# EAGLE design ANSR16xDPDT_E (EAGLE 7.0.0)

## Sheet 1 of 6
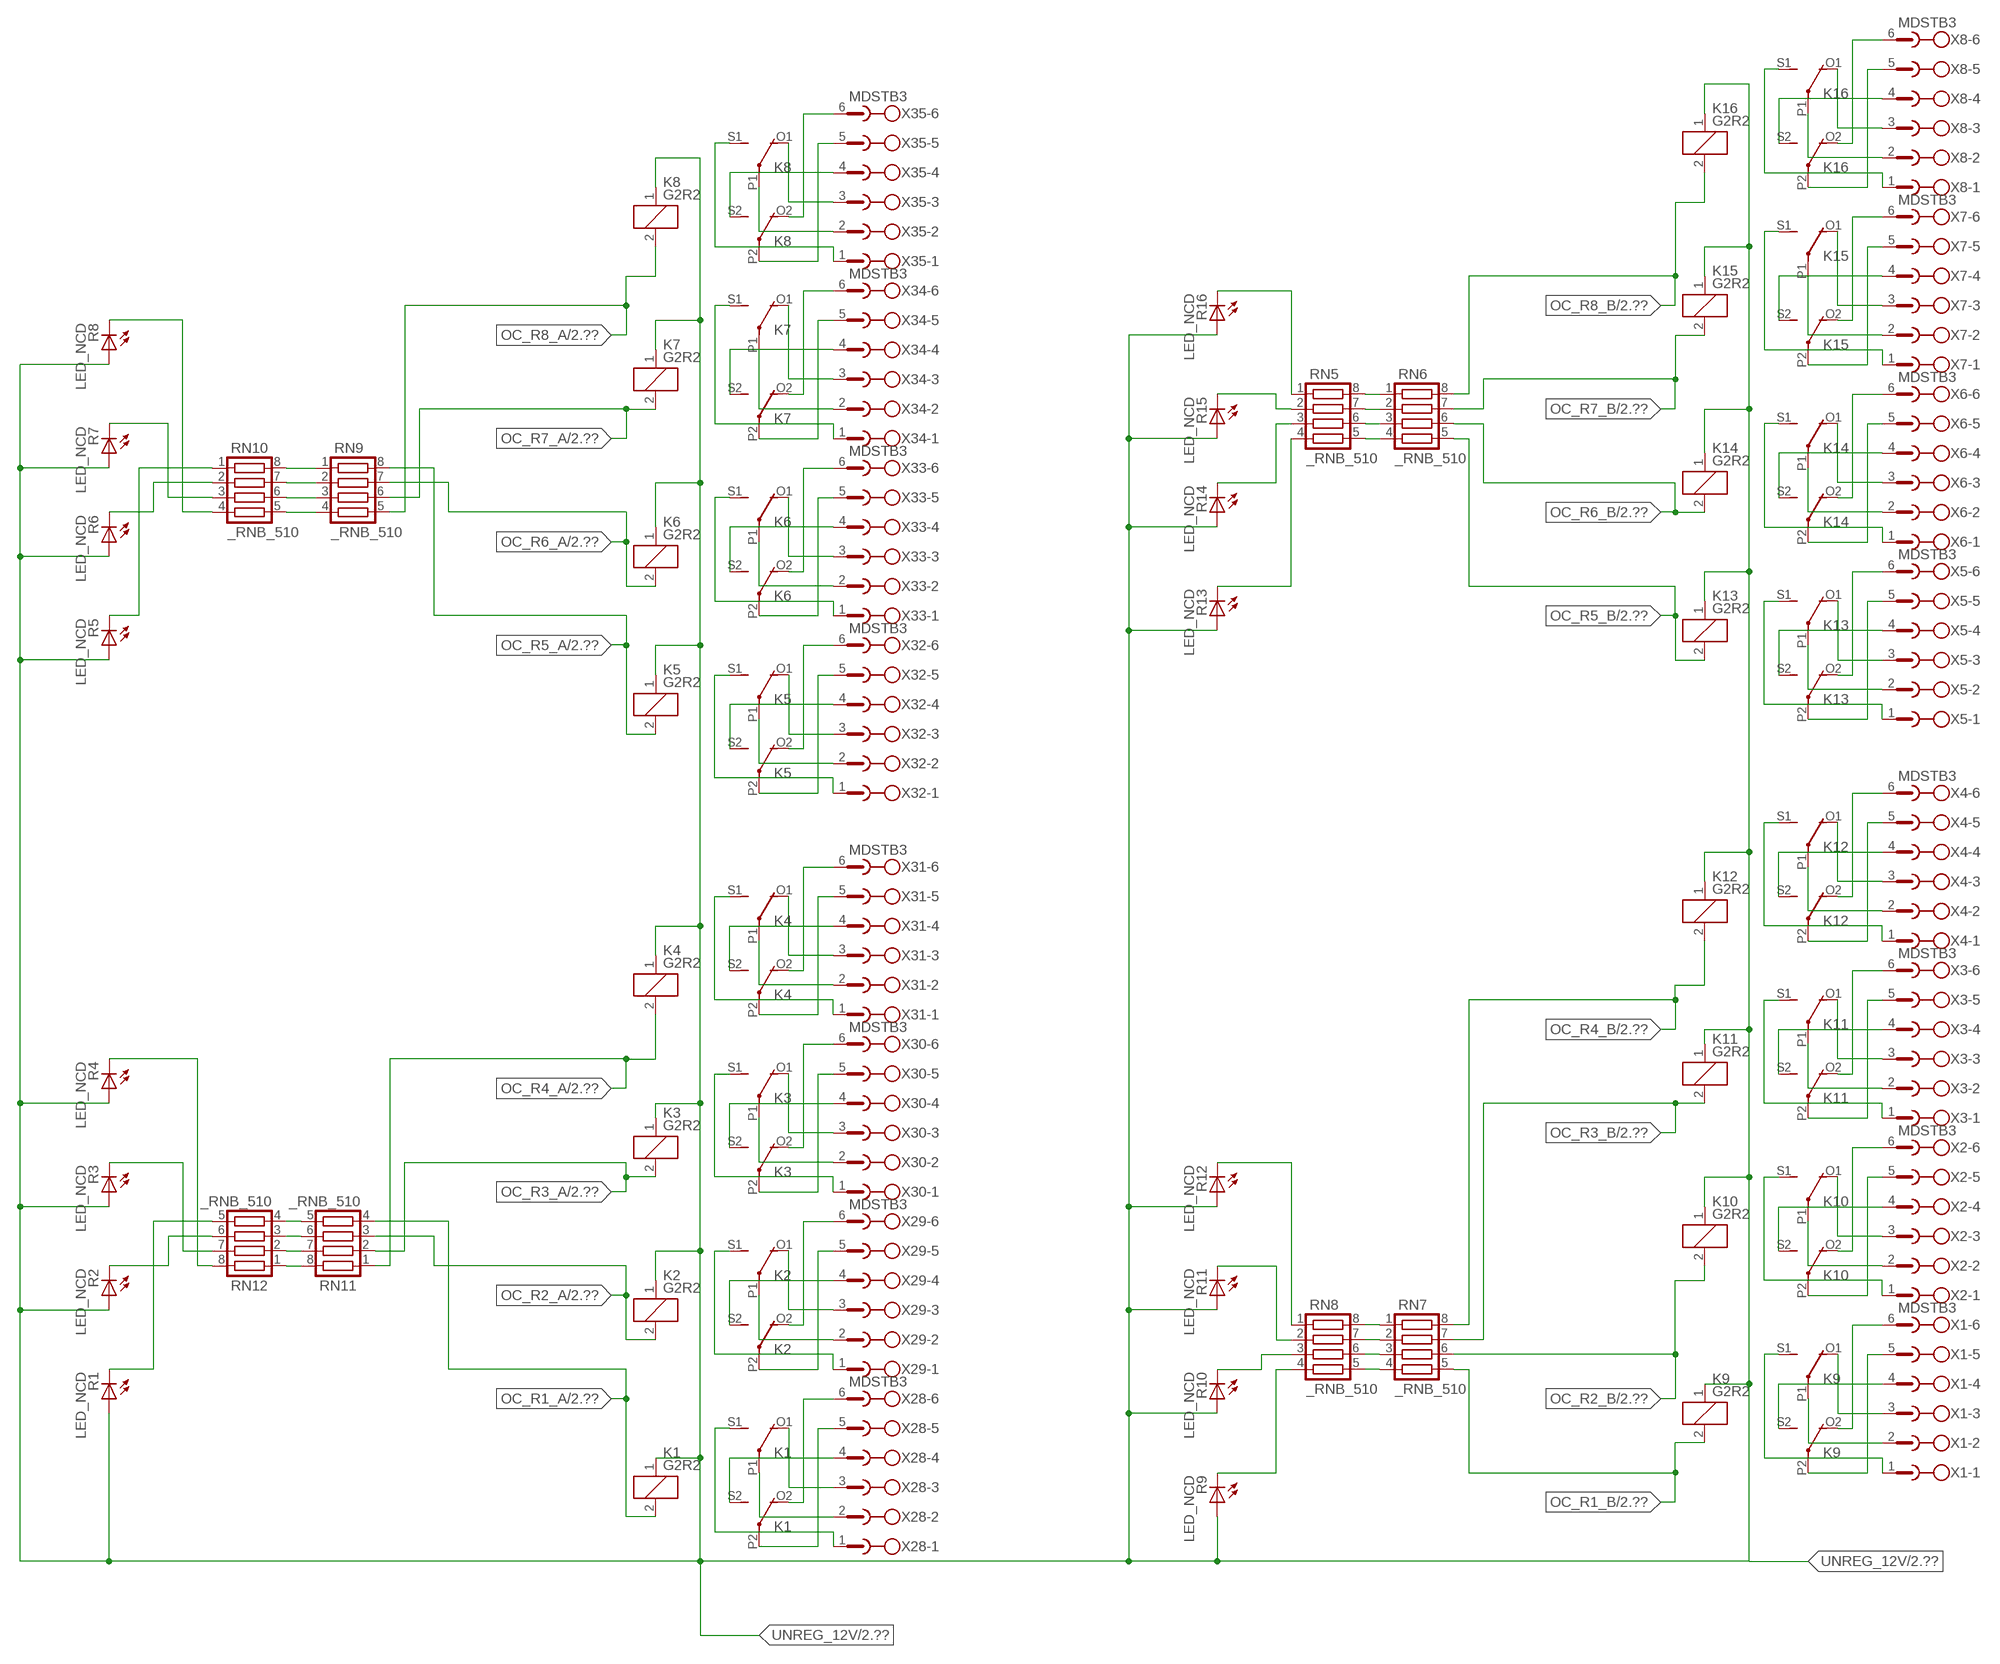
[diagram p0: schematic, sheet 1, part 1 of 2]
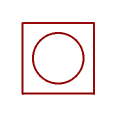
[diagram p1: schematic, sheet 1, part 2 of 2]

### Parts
K1  G2R2  [G2R2]
K2  G2R2  [G2R2]
K3  G2R2  [G2R2]
K4  G2R2  [G2R2]
K5  G2R2  [G2R2]
K6  G2R2  [G2R2]
K7  G2R2  [G2R2]
K8  G2R2  [G2R2]
K9  G2R2  [G2R2]
K10  G2R2  [G2R2]
K11  G2R2  [G2R2]
K12  G2R2  [G2R2]
K13  G2R2  [G2R2]
K14  G2R2  [G2R2]
K15  G2R2  [G2R2]
K16  G2R2  [G2R2]
R1  LED_NCD  [CHIPLED_0603]
R2  LED_NCD  [CHIPLED_0603]
R3  LED_NCD  [CHIPLED_0603]
R4  LED_NCD  [CHIPLED_0603]
R5  LED_NCD  [CHIPLED_0603]
R6  LED_NCD  [CHIPLED_0603]
R7  LED_NCD  [CHIPLED_0603]
R8  LED_NCD  [CHIPLED_0603]
R9  LED_NCD  [CHIPLED_0603]
R10  LED_NCD  [CHIPLED_0603]
R11  LED_NCD  [CHIPLED_0603]
R12  LED_NCD  [CHIPLED_0603]
R13  LED_NCD  [CHIPLED_0603]
R14  LED_NCD  [CHIPLED_0603]
R15  LED_NCD  [CHIPLED_0603]
R16  LED_NCD  [CHIPLED_0603]
RN5  _RNB_510  [RNB]
RN6  _RNB_510  [RNB]
RN7  _RNB_510  [RNB]
RN8  _RNB_510  [RNB]
RN9  _RNB_510  [RNB]
RN10  _RNB_510  [RNB]
RN11  _RNB_510  [RNB]
RN12  _RNB_510  [RNB]
U$1  PCB_MOUNTING_HOLE  [PCB_MOUNTING_HOLE]
X1  MDSTB3  [MDSTB3]
X2  MDSTB3  [MDSTB3]
X3  MDSTB3  [MDSTB3]
X4  MDSTB3  [MDSTB3]
X5  MDSTB3  [MDSTB3]
X6  MDSTB3  [MDSTB3]
X7  MDSTB3  [MDSTB3]
X8  MDSTB3  [MDSTB3]
X28  MDSTB3  [MDSTB3]
X29  MDSTB3  [MDSTB3]
X30  MDSTB3  [MDSTB3]
X31  MDSTB3  [MDSTB3]
X32  MDSTB3  [MDSTB3]
X33  MDSTB3  [MDSTB3]
X34  MDSTB3  [MDSTB3]
X35  MDSTB3  [MDSTB3]

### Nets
N$1: K9.P2(3:COM) X1.5
N$2: K9.O2(3:NC) X1.6
N$3: K9.S2(3:NO) X1.4
N$4: K9.P1(2:COM) X1.2
N$5: K9.O1(2:NC) X1.3
N$6: K9.S1(2:NO) X1.1
N$7: K10.P2(3:COM) X2.5
N$8: K10.O2(3:NC) X2.6
N$9: K10.S2(3:NO) X2.4
N$10: K10.S1(2:NO) X2.1
N$11: K10.P1(2:COM) X2.2
N$12: K10.O1(2:NC) X2.3
N$13: K11.P2(3:COM) X3.5
N$14: K11.O2(3:NC) X3.6
N$15: K12.P2(3:COM) X4.5
N$16: K12.O2(3:NC) X4.6
N$17: K11.S2(3:NO) X3.4
N$18: K12.S2(3:NO) X4.4
N$19: K11.O1(2:NC) X3.3
N$20: K12.O1(2:NC) X4.3
N$21: K12.P1(2:COM) X4.2
N$22: K11.P1(2:COM) X3.2
N$23: K11.S1(2:NO) X3.1
N$24: K12.S1(2:NO) X4.1
N$25: K13.O2(3:NC) X5.6
N$26: K13.P2(3:COM) X5.5
N$27: K13.S2(3:NO) X5.4
N$28: K13.P1(2:COM) X5.2
N$29: K13.S1(2:NO) X5.1
N$30: K13.O1(2:NC) X5.3
N$31: K14.P2(3:COM) X6.5
N$32: K14.O2(3:NC) X6.6
N$33: K14.P1(2:COM) X6.2
N$34: K14.S1(2:NO) X6.1
N$35: K15.P1(2:COM) X7.2
N$36: K16.P1(2:COM) X8.2
N$37: K16.P2(3:COM) X8.5
N$38: K16.O2(3:NC) X8.6
N$39: K14.O1(2:NC) X6.3
N$40: K16.O1(2:NC) X8.3
N$41: K15.O1(2:NC) X7.3
N$42: K15.O2(3:NC) X7.6
N$43: K15.P2(3:COM) X7.5
N$44: K14.S2(3:NO) X6.4
N$45: K15.S2(3:NO) X7.4
N$46: K15.S1(2:NO) X7.1
N$47: K16.S1(2:NO) X8.1
N$48: K16.S2(3:NO) X8.4
N$203: K1.P2(3:COM) X28.5
N$204: K1.O2(3:NC) X28.6
N$205: K1.S2(3:NO) X28.4
N$206: K1.P1(2:COM) X28.2
N$207: K1.O1(2:NC) X28.3
N$208: K1.S1(2:NO) X28.1
N$209: K2.P2(3:COM) X29.5
N$210: K2.O2(3:NC) X29.6
N$211: K2.S2(3:NO) X29.4
N$212: K2.S1(2:NO) X29.1
N$213: K2.P1(2:COM) X29.2
N$214: K2.O1(2:NC) X29.3
N$215: K3.P2(3:COM) X30.5
N$216: K3.O2(3:NC) X30.6
N$217: K4.P2(3:COM) X31.5
N$218: K4.O2(3:NC) X31.6
N$219: K3.S2(3:NO) X30.4
N$220: K4.S2(3:NO) X31.4
N$221: K3.O1(2:NC) X30.3
N$222: K4.O1(2:NC) X31.3
N$223: K4.P1(2:COM) X31.2
N$224: K3.P1(2:COM) X30.2
N$225: K3.S1(2:NO) X30.1
N$226: K4.S1(2:NO) X31.1
N$304: K5.O2(3:NC) X32.6
N$305: K5.P2(3:COM) X32.5
N$306: K5.S2(3:NO) X32.4
N$307: K5.P1(2:COM) X32.2
N$308: K5.S1(2:NO) X32.1
N$309: K5.O1(2:NC) X32.3
N$310: K6.P2(3:COM) X33.5
N$311: K6.O2(3:NC) X33.6
N$312: K6.P1(2:COM) X33.2
N$313: K6.S1(2:NO) X33.1
N$314: K7.P1(2:COM) X34.2
N$315: K8.P1(2:COM) X35.2
N$316: K8.P2(3:COM) X35.5
N$317: K8.O2(3:NC) X35.6
N$318: K6.O1(2:NC) X33.3
N$319: K8.O1(2:NC) X35.3
N$320: K7.O1(2:NC) X34.3
N$321: K7.O2(3:NC) X34.6
N$322: K7.P2(3:COM) X34.5
N$323: K6.S2(3:NO) X33.4
N$324: K7.S2(3:NO) X34.4
N$325: K7.S1(2:NO) X34.1
N$326: K8.S1(2:NO) X35.1
N$327: K8.S2(3:NO) X35.4
N$441: R16.C RN5.1
N$442: RN7.2 RN8.7
N$443: RN7.3 RN8.6
N$444: RN7.4 RN8.5
N$445: R15.C RN5.2
N$447: R13.C RN5.4
N$448: RN5.5 RN6.4
N$449: RN7.1 RN8.8
N$450: R12.C RN8.1
N$451: RN5.6 RN6.3
N$452: R11.C RN8.2
N$453: RN5.7 RN6.2
N$454: RN5.8 RN6.1
N$458: R14.C RN5.3
N$459: R10.C RN8.3
N$463: RN11.5 RN12.4
N$470: R9.C RN8.4
N$473: R1.C RN12.5
N$474: RN11.6 RN12.3
N$475: R2.C RN12.6
N$476: R3.C RN12.7
N$477: RN9.4 RN10.5
N$478: RN9.3 RN10.6
N$479: RN9.2 RN10.7
N$480: RN9.1 RN10.8
N$481: RN11.7 RN12.2
N$482: R5.C RN10.1
N$483: R4.C RN12.8
N$484: R7.C RN10.3
N$485: R8.C RN10.4
N$486: R6.C RN10.2
N$500: RN11.8 RN12.1
OC_R1_A: K1.2(1:C2) RN11.4 ; also sheet 2
OC_R1_B: K9.2(1:C2) RN7.5 ; also sheet 2
OC_R2_A: K2.2(1:C2) RN11.3 ; also sheet 2
OC_R2_B: K10.2(1:C2) RN7.6 ; also sheet 2
OC_R3_A: K3.2(1:C2) RN11.2 ; also sheet 2
OC_R3_B: K11.2(1:C2) RN7.7 ; also sheet 2
OC_R4_A: K4.2(1:C2) RN11.1 ; also sheet 2
OC_R4_B: K12.2(1:C2) RN7.8 ; also sheet 2
OC_R5_A: K5.2(1:C2) RN9.8 ; also sheet 2
OC_R5_B: K13.2(1:C2) RN6.5 ; also sheet 2
OC_R6_A: K6.2(1:C2) RN9.7 ; also sheet 2
OC_R6_B: K14.2(1:C2) RN6.6 ; also sheet 2
OC_R7_A: K7.2(1:C2) RN9.6 ; also sheet 2
OC_R7_B: K15.2(1:C2) RN6.7 ; also sheet 2
OC_R8_A: K8.2(1:C2) RN9.5 ; also sheet 2
OC_R8_B: K16.2(1:C2) RN6.8 ; also sheet 2
UNREG_12V: K1.1(1:C1) K2.1(1:C1) K3.1(1:C1) K4.1(1:C1) K5.1(1:C1) K6.1(1:C1) K7.1(1:C1) K8.1(1:C1) K9.1(1:C1) K10.1(1:C1) K11.1(1:C1) K12.1(1:C1) K13.1(1:C1) K14.1(1:C1) K15.1(1:C1) K16.1(1:C1) R1.A R2.A R3.A R4.A R5.A R6.A R7.A R8.A R9.A R10.A R11.A R12.A R13.A R14.A R15.A R16.A ; also sheet 2,3

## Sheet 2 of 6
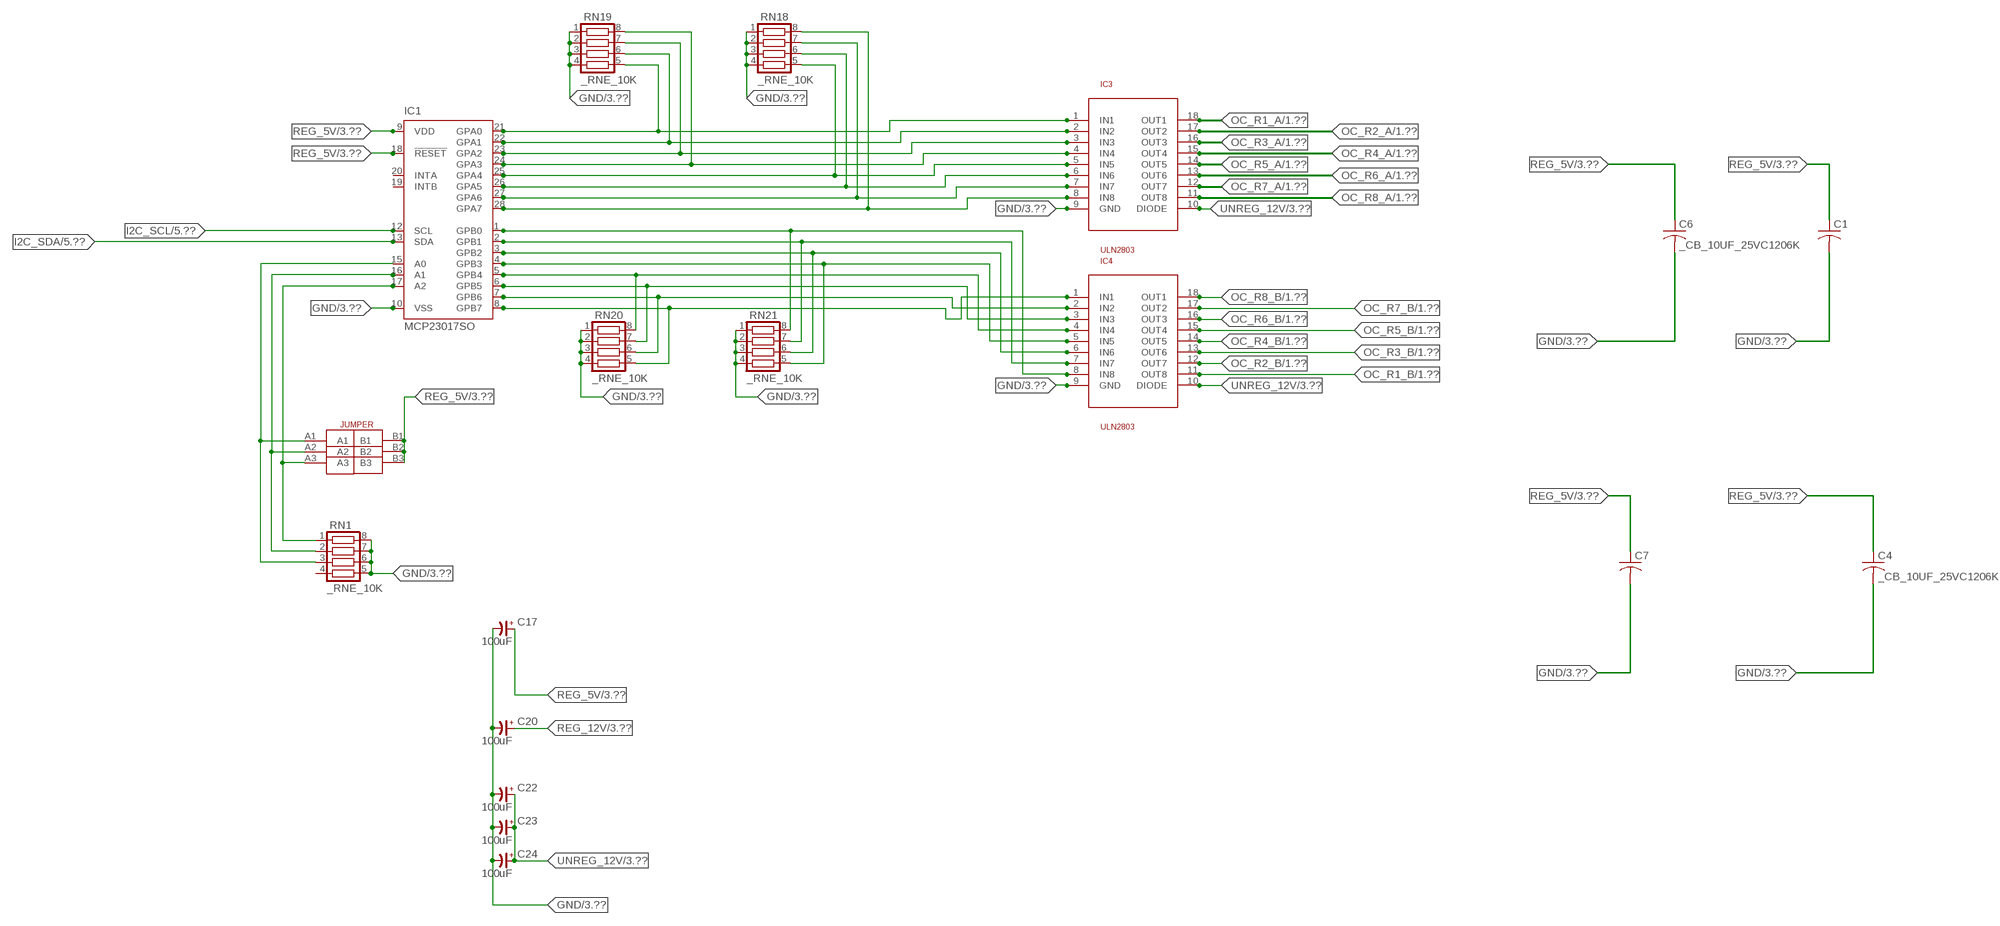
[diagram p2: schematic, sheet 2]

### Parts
C1  _CA_.10UF_50VC1206K  [_CA_.1UF_50V]
C4  _CB_10UF_25VC1206K  [_CB_10UF_25V]
C6  _CB_10UF_25VC1206K  [_CB_10UF_25V]
C7  _CA_.10UF_50VC1206K  [_CA_.1UF_50V]
C17  100uF  CP-E-025X060  [E-025X060]
C20  100uF  CP-E-025X060  [E-025X060]
C22  100uF  CP-E-025X060  [E-025X060]
C23  100uF  CP-E-025X060  [E-025X060]
C24  100uF  CP-E-025X060  [E-025X060]
IC1  MCP23017SO  [SO28W]
IC3  ULN2803  [SO18L]
IC4  ULN2803  [SO18L]
JP1  JUMPER_3X2  [JUMPER_3X2]
RN1  _RNE_10K  [RNE]
RN18  _RNE_10K  [RNE]
RN19  _RNE_10K  [RNE]
RN20  _RNE_10K  [RNE]
RN21  _RNE_10K  [RNE]

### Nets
GND: C1.2 C4.2 C6.2 C7.2 C17.- C20.- C22.- C23.- C24.- IC1.10(VSS) IC3.9(GND) IC4.9(GND) RN1.5 RN1.6 RN1.7 RN1.8 RN18.1 RN18.2 RN18.3 RN18.4 RN19.1 RN19.2 RN19.3 RN19.4 RN20.1 RN20.2 RN20.3 RN20.4 RN21.1 RN21.2 RN21.3 RN21.4 ; also sheet 3,4,5,6
I2C_SCL: IC1.12(SCL) ; also sheet 5,6
I2C_SDA: IC1.13(SDA) ; also sheet 5,6
N$49: IC1.15(A0) JP1.A1 RN1.3
N$405: IC1.21(GPA0) IC3.1(IN1) RN19.5
N$406: IC1.25(GPA4) IC3.5(IN5) RN18.5
N$407: IC1.26(GPA5) IC3.6(IN6) RN18.6
N$408: IC1.16(A1) JP1.A2 RN1.2
N$409: IC1.22(GPA1) IC3.2(IN2) RN19.6
N$410: IC1.23(GPA2) IC3.3(IN3) RN19.7
N$411: IC1.24(GPA3) IC3.4(IN4) RN19.8
N$416: IC1.1(GPB0) IC4.8(IN8) RN21.8
N$417: IC1.2(GPB1) IC4.7(IN7) RN21.7
N$418: IC1.3(GPB2) IC4.6(IN6) RN21.6
N$419: IC1.4(GPB3) IC4.5(IN5) RN21.5
N$420: IC1.5(GPB4) IC4.4(IN4) RN20.8
N$421: IC1.6(GPB5) IC4.3(IN3) RN20.7
N$422: IC1.7(GPB6) IC4.2(IN2) RN20.6
N$423: IC1.8(GPB7) IC4.1(IN1) RN20.5
N$498: IC1.17(A2) JP1.A3 RN1.1
N$525: IC1.27(GPA6) IC3.7(IN7) RN18.7
N$526: IC1.28(GPA7) IC3.8(IN8) RN18.8
OC_R1_A: IC3.18(OUT1) ; also sheet 1
OC_R1_B: IC4.11(OUT8) ; also sheet 1
OC_R2_A: IC3.17(OUT2) ; also sheet 1
OC_R2_B: IC4.12(OUT7) ; also sheet 1
OC_R3_A: IC3.16(OUT3) ; also sheet 1
OC_R3_B: IC4.13(OUT6) ; also sheet 1
OC_R4_A: IC3.15(OUT4) ; also sheet 1
OC_R4_B: IC4.14(OUT5) ; also sheet 1
OC_R5_A: IC3.14(OUT5) ; also sheet 1
OC_R5_B: IC4.15(OUT4) ; also sheet 1
OC_R6_A: IC3.13(OUT6) ; also sheet 1
OC_R6_B: IC4.16(OUT3) ; also sheet 1
OC_R7_A: IC3.12(OUT7) ; also sheet 1
OC_R7_B: IC4.17(OUT2) ; also sheet 1
OC_R8_A: IC3.11(OUT8) ; also sheet 1
OC_R8_B: IC4.18(OUT1) ; also sheet 1
REG_5V: C1.1 C4.1 C6.1 C7.1 C17.+ IC1.9(VDD) IC1.18(!RESET) JP1.B1 JP1.B2 JP1.B3 ; also sheet 3,4,5,6
REG_12V: C20.+ ; also sheet 3,4
UNREG_12V: C22.+ C23.+ C24.+ IC3.10(DIODE) IC4.10(DIODE) ; also sheet 1,3
Unconnected: IC1.19(INTB) IC1.20(INTA) RN1.4

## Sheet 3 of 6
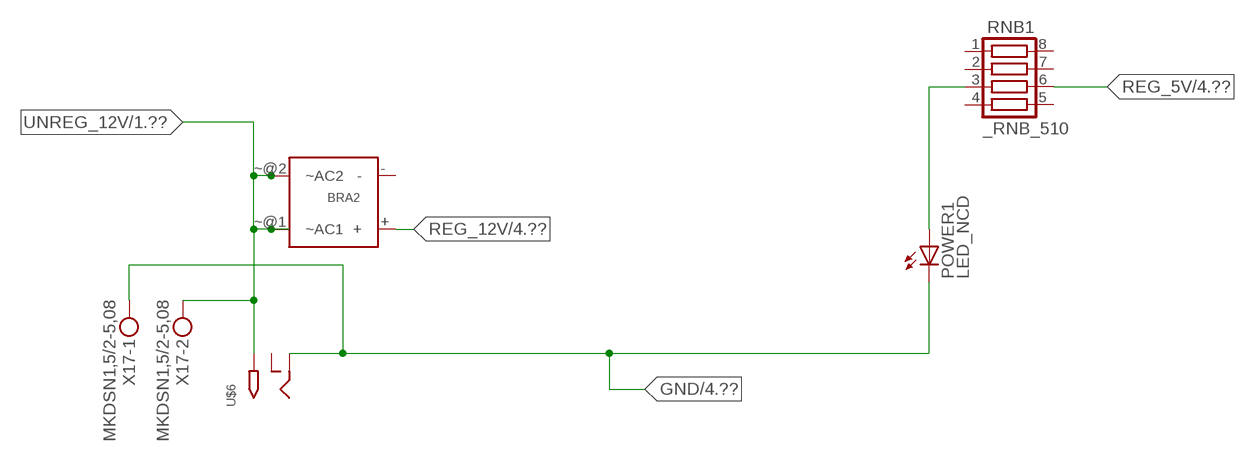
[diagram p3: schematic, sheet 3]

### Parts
BRA2  MB2S_  [MB2S]
POWER1  LED_NCD  [CHIPLED_0603]
RNB1  _RNB_510  [RNB]
U$6  2.1MMJACK  [PJ-102A]
X17  MKDSN1,5/2-5,08  [MKDSN1,5/2-5,08]

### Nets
GND: POWER1.C U$6.RING X17.1 ; also sheet 2,4,5,6
N$99: POWER1.A RNB1.3
REG_5V: RNB1.6 ; also sheet 2,4,5,6
REG_12V: BRA2.+ ; also sheet 2,4
UNREG_12V: BRA2.~@1(~AC1) BRA2.~@2(~AC2) U$6.TIP X17.2 ; also sheet 1,2
Unconnected: BRA2.- RNB1.1 RNB1.2 RNB1.4 RNB1.5 RNB1.7 RNB1.8 U$6.RING_SW

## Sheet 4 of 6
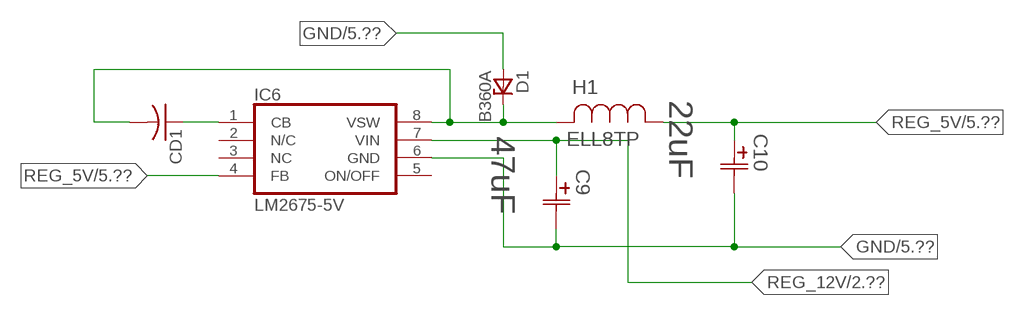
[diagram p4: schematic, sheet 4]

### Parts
C9  47uF  490-5463-6-NDCAP  [C2917(7343)-Y]
C10  22uF  490-5463-6-NDCAP  [C2917(7343)-Y]
CD1  _CD_10NF_50VC1206K  [_CD_10NF_50V]
D1  B360A  [DO214AC_ZENER]
H1  ELL8TP  [IND_ELL8TP]
IC6  LM2675-5V  LM2675  [SO-8]

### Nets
GND: C9.2(C2) C10.2(C2) D1.A IC6.6(GND) ; also sheet 2,3,5,6
N$100: CD1.2 D1.C H1.2 IC6.8(VSW)
N$101: CD1.1 IC6.1(CB)
REG_5V: C10.1(C1) H1.1 IC6.4(FB) ; also sheet 2,3,5,6
REG_12V: C9.1(C1) IC6.7(VIN) ; also sheet 2,3
Unconnected: IC6.2(N/C) IC6.5(ON/OFF)

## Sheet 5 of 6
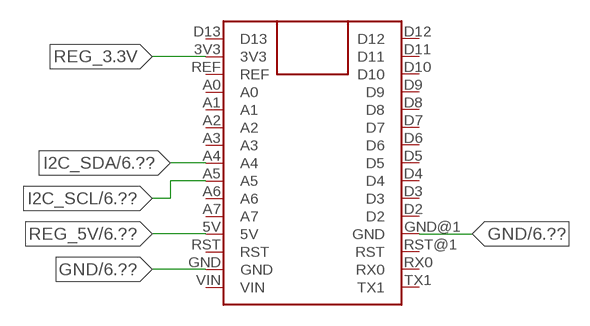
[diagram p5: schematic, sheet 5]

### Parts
FOR_NANO  ARDUINO_NANO  [ARDUINO_NANO]

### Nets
GND: FOR_NANO.GND FOR_NANO.GND@1(GND) ; also sheet 2,3,4,6
I2C_SCL: FOR_NANO.A5 ; also sheet 2,6
I2C_SDA: FOR_NANO.A4 ; also sheet 2,6
REG_3.3V: FOR_NANO.3V3
REG_5V: FOR_NANO.5V ; also sheet 2,3,4,6
Unconnected: FOR_NANO.A0 FOR_NANO.A1 FOR_NANO.A2 FOR_NANO.A3 FOR_NANO.A6 FOR_NANO.A7 FOR_NANO.D2 FOR_NANO.D3 FOR_NANO.D4 FOR_NANO.D5 FOR_NANO.D6 FOR_NANO.D7 FOR_NANO.D8 FOR_NANO.D9 FOR_NANO.D10 FOR_NANO.D11 FOR_NANO.D12 FOR_NANO.D13 FOR_NANO.REF FOR_NANO.RST FOR_NANO.RST@1(RST) FOR_NANO.RX0 FOR_NANO.TX1 FOR_NANO.VIN

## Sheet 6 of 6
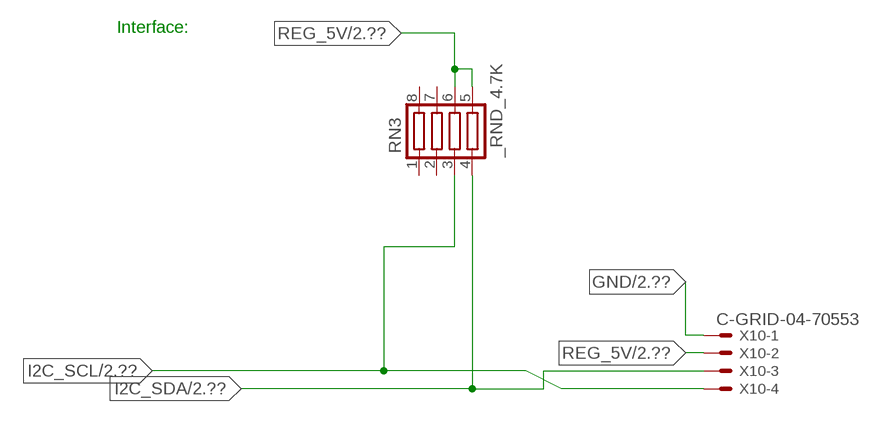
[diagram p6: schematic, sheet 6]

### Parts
RN3  _RND_4.7K  [RND]
X10  C-GRID-04-70553  [70553-04]

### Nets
GND: X10.1 ; also sheet 2,3,4,5
I2C_SCL: RN3.3 X10.4 ; also sheet 2,5
I2C_SDA: RN3.4 X10.3 ; also sheet 2,5
REG_5V: RN3.5 RN3.6 X10.2 ; also sheet 2,3,4,5
Unconnected: RN3.1 RN3.2 RN3.7 RN3.8

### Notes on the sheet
- Interface:

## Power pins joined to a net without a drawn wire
NC: IC6.3(NC)

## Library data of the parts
BRA2 = NCD_ULTIMATE_LIBRARY:MB2S: Bridge Rectifier BRA MB2S 200V 500ma Digikey MB2S-TPMSTR-ND/MB2S-TP
C1 C7 = NCD_ULTIMATE_LIBRARY:_CA_.10UF_50V: Capacitor .1uF SMT
C4 C6 = NCD_ULTIMATE_LIBRARY:_CB_10UF_25V: Capacitor 10uF SMT
C9 C10 = NCD_ULTIMATE_bhaskar:490-5463-6-ND: NCD CAP
C17 C20 C22-C24 = NCD_ULTIMATE_LIBRARY:CP-: Capacitors All Kinds POLARIZED CAP
CD1 = NCD_ULTIMATE_LIBRARY:_CD_10NF_50V: Capacitor 10nF SMT
D1 = NCD_ULTIMATE_bhaskar:B360A: NCD DIODE B350A/B360A
FOR_NANO = NCD_ULTIMATE_CONNECTORS:ARDUINO_NANO
H1 = NCD_ULTIMATE_bhaskar:ELL8TP: NCD coil
IC1 = NCD_ULTIMATE_LIBRARY:MCP23017: Semiconductor Port Expander I/O 16-Bit I2C http://ww1.microchip.com/downloads/en/DeviceDoc/21952a.pdf Source: http://ww1.microchip.com/downloads/en/DeviceDoc/21952a.pdf
IC3 IC4 = NCD_ULTIMATE_LIBRARY:ULN2803: Semiconductor 8 O.C. N-Channel Transistor Driver Digikey ULN2803AFWGCELTR-ND/ULN2803AFWG,C,EL
IC6 = NCD_ULTIMATE_bhaskar:LM2675: LM2675 NCD http://www.ti.com/lit/ds/symlink/lm2675.pdf
JP1 = NCD_ULTIMATE_CONNECTORS:JUMPER_3X2
K1-K16 = NCD_ULTIMATE_LIBRARY:G2R2: RELAY 2 x switch, Omron
POWER1 R1-R16 = NCD_ULTIMATE_bhaskar:LED_NCD
RN1 RN18-RN21 = NCD_ULTIMATE_LIBRARY:_RNE_10K: Resistor Array RNE SMT 10K x 4 Single Resistor Source: http://www.ctscorp.com/components/Datasheets/CTSChipArrayDs.pdf Digikey 742C083103JPTR-ND/742C083103JP; OC_FARNELL: unknown; OC_NEWARK: unknown
RN3 = NCD_ULTIMATE_LIBRARY:_RND_4.7K: Resistor Array RND SMT 4.7K x 4 Single Resistor Source: http://www.ctscorp.com/components/Datasheets/CTSChipArrayDs.pdf Digikey 742C083472JPTR-ND/742C083472JP; OC_FARNELL: unknown; OC_NEWARK: unknown
RN5-RN12 RNB1 = NCD_ULTIMATE_LIBRARY:_RNB_510: Resistor Array RNB SMT 510 x 4 Single Resistor Source: http://www.ctscorp.com/components/Datasheets/CTSChipArrayDs.pdf Digikey 742C083511JPTR-ND/ 742C083511JP; OC_FARNELL: unknown; OC_NEWARK: unknown
U$1 = NCD_ULTIMATE_CONNECTORS:PCB_MOUNTING_HOLE
U$6 = NCD_ULTIMATE_CONNECTORS:2.1MMJACK: 2.1mm x 5.5mm DC jack with internal switch. Digikey part #PJ-102A, 4UCON part #05537 By microbuilder.eu
X1-X8 X28-X35 = NCD_ULTIMATE_LIBRARY:MDSTB3: PHOENIX
X10 = NCD_ULTIMATE_CONNECTORS:C-GRID-04: CONNECTOR 4-Pos I2C wire to board 2.54 mm (0.100") pitch header Digikey WM1342-ND/0015912045; OC_FARNELL: unknown; OC_NEWARK: unknown
X17 = NCD_ULTIMATE_CONNECTORS:MKDSN1,5/2-5,08: MKDSN 1,5/ 2-5,08 Printklemme

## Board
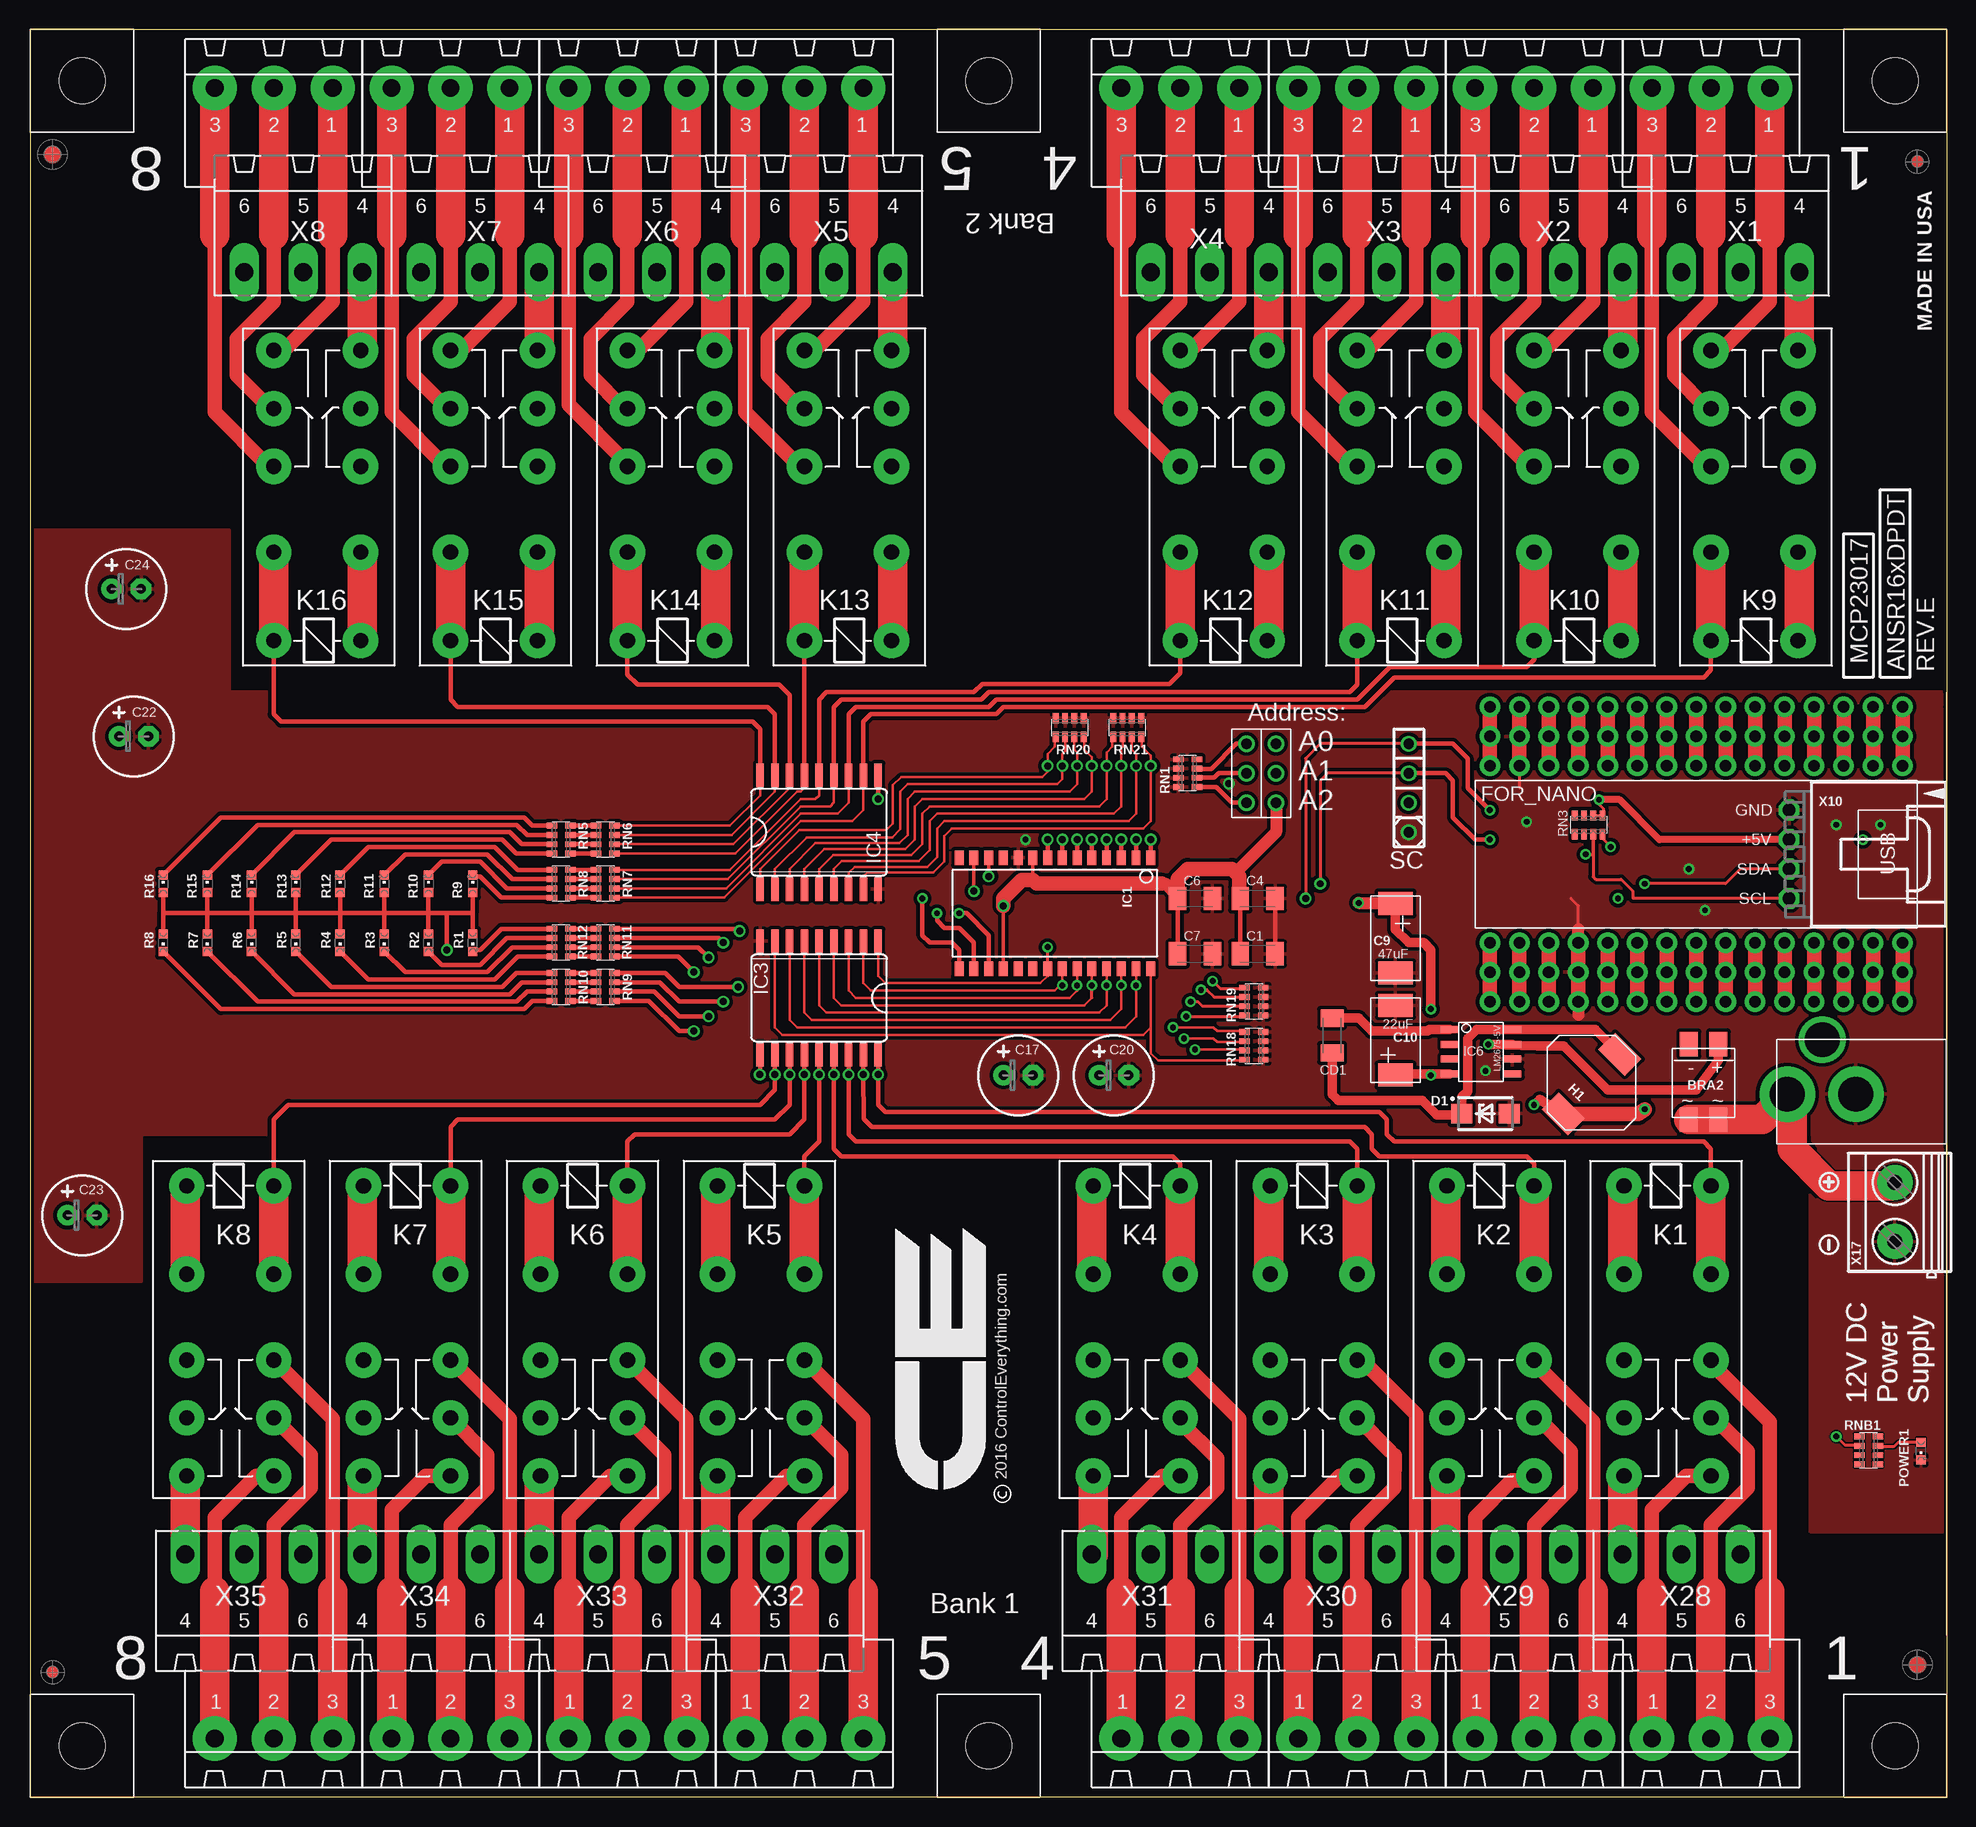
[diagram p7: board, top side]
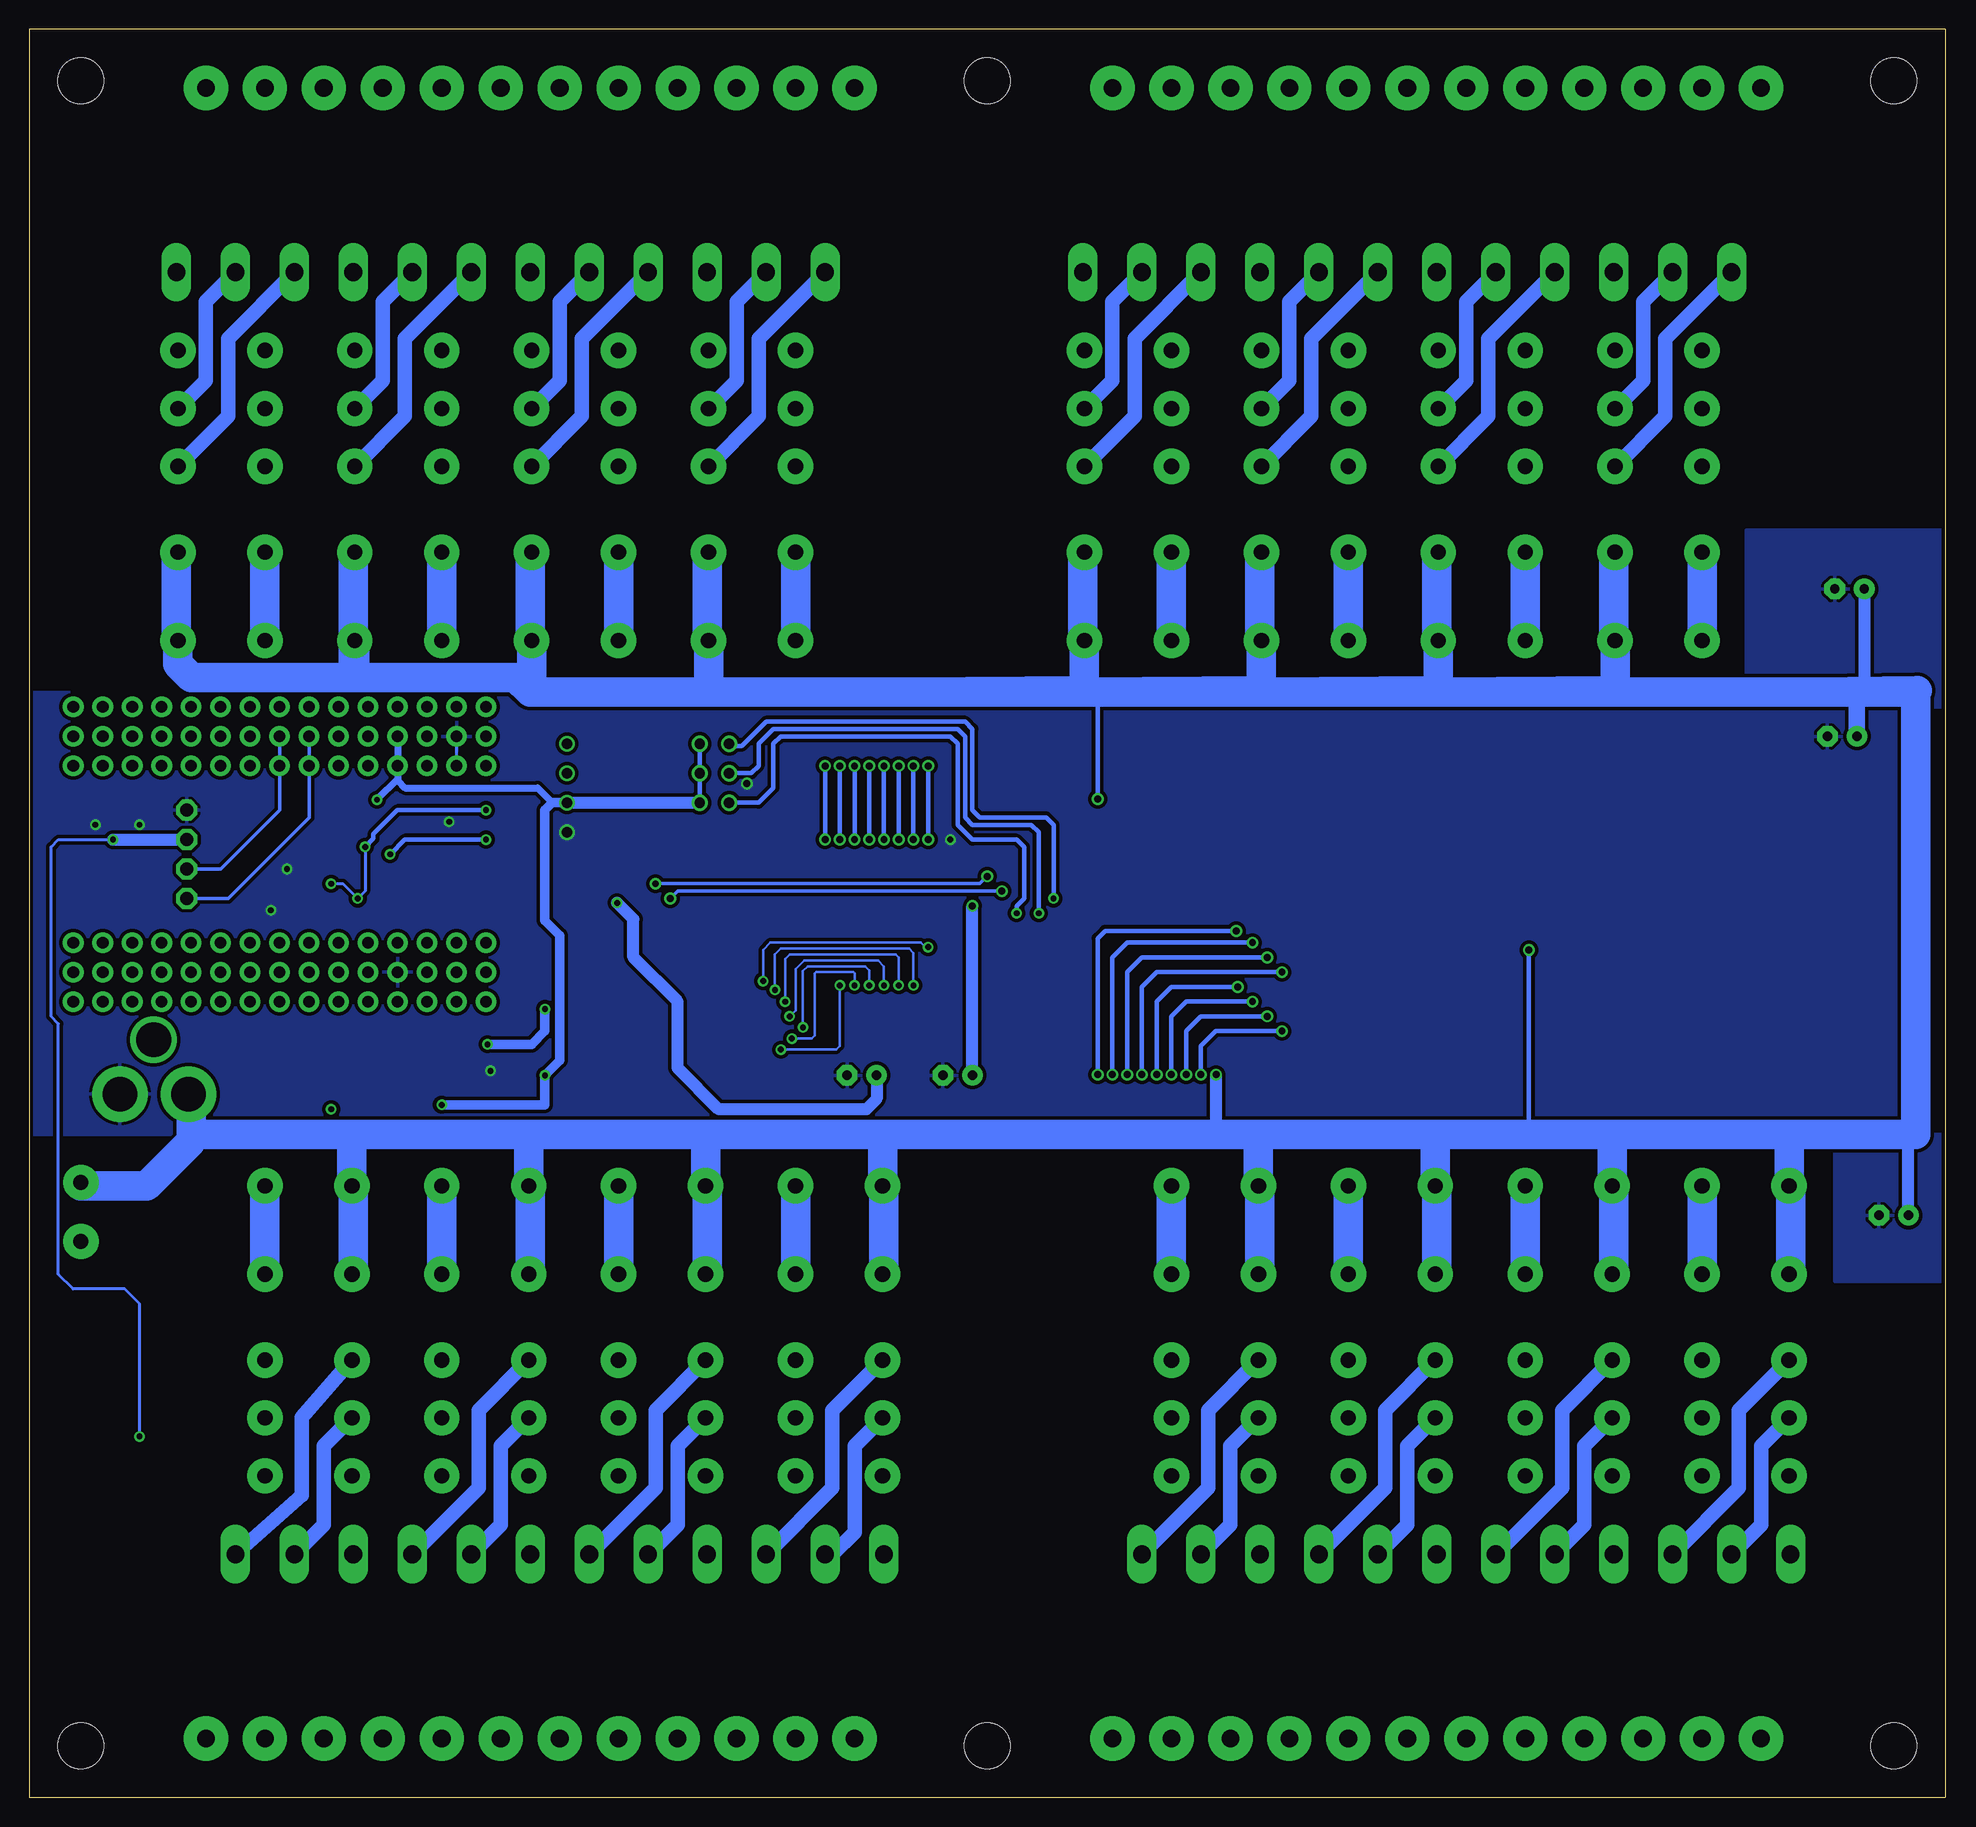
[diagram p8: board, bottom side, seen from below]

Size 165.1 x 152.41 mm. Coordinates in mm from the lower left corner, seen from the top.
Outline: 165.08,0 165.08,152.41 0,152.41 0,0.01 165.1,0.01
Outline: 165.08,93.99 165.08,13.97
Outline: 165.08,95.26 165.08,14.6
Outline: 165.1,95.26 165.1,37.48
Copper layers (1*16): Top 0.035mm / dielectric 1.5mm / Bottom 0.035mm
Design rules "default": minimum track width 5mil, minimum drill 24mil, track to track 5mil, track to pad 5mil, pad to pad 5mil, via to via 5mil, smd to smd 5mil, copper to edge 10mil, drill to drill 8mil, minimum pad ring 10mil, minimum via ring 8mil, stop-mask expansion 2mil, vias tented up to drill 0mil, thermal gap 10mil

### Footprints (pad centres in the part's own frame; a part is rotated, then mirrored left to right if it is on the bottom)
MB2S = smd 1.55 x 2.1: + 0,-6.5; - 2.54,-6.5; ~@1 0,0; ~@2 2.54,0
_CA_.1UF_50V = smd 1.5 x 2: 1 -1.5,0; 2 1.5,0
_CB_10UF_25V = smd 1.5 x 2: 1 -1.5,0; 2 1.5,0
C2917(7343)-Y = smd 2 x 3: 1 -3,0; 2 3,0
E-025X060 = drill 0.813 pad 1.778: + -1.27,0 | drill 0.813 pad 1.778 octagon: - 1.27,0
_CD_10NF_50V = smd 1.5 x 2: 1 -1.5,0; 2 1.5,0
DO214AC_ZENER = smd 1.8 x 1.7: A 2.05,0; C -2.05,0
ARDUINO_NANO = drill 1 pad 1.778: 3V1 -2.54,-2.54; 3V3 0,-2.54; 5V 0,-27.94; 5V1 -2.54,-27.94; A0 0,-7.62; A1 0,-10.16; A2 0,-12.7; A3 0,-15.24; A4 0,-17.78; A5 0,-20.32; A6 0,-22.86; A7 0,-25.4; A8 -2.54,-7.62; A9 -2.54,-10.16; A10 -2.54,-12.7; A11 -2.54,-15.24; A12 -2.54,-17.78; A13 -2.54,-20.32; A14 -2.54,-22.86; A15 -2.54,-25.4; D1 -2.54,0; D2 20.32,-25.4; D3 20.32,-22.86; D4 20.32,-20.32; D5 20.32,-17.78; D6 20.32,-15.24; D7 20.32,-12.7; D8 20.32,-10.16; D9 20.32,-7.62; D10 20.32,-5.08; D11 20.32,-2.54; D12 20.32,0; D13 0,0; D14 22.86,0; D15 22.86,-2.54; D16 22.86,-5.08; D17 22.86,-7.62; D18 22.86,-10.16; D19 22.86,-12.7; D20 22.86,-15.24; D21 22.86,-17.78; D22 22.86,-20.32; D23 22.86,-22.86; D24 22.86,-25.4; GND 0,-33.02; GND1 -2.54,-33.02; GND@1 20.32,-27.94; GND@2 22.86,-27.94; P$16 2.54,0; P$17 2.54,-2.54; P$18 2.54,-5.08; P$19 2.54,-7.62; P$20 2.54,-10.16; P$21 2.54,-12.7; P$22 2.54,-15.24; P$23 2.54,-17.78; P$24 2.54,-20.32; P$25 2.54,-22.86; P$26 2.54,-25.4; P$27 2.54,-27.94; P$28 2.54,-30.48; P$29 2.54,-33.02; P$30 2.54,-35.56; P$31 17.78,0; P$32 17.78,-2.54; P$33 17.78,-5.08; P$34 17.78,-7.62; P$35 17.78,-10.16; P$36 17.78,-12.7; P$37 17.78,-15.24; P$38 17.78,-17.78; P$39 17.78,-20.32; P$40 17.78,-22.86; P$41 17.78,-25.4; P$42 17.78,-27.94; P$43 17.78,-30.48; P$44 17.78,-33.02; P$45 17.78,-35.56; REF 0,-5.08; REF1 -2.54,-5.08; RST 0,-30.48; RST1 -2.54,-30.48; RST@1 20.32,-30.48; RST@2 22.86,-30.48; RX0 20.32,-33.02; RX1 22.86,-33.02; TX1 20.32,-35.56; TX2 22.86,-35.56; VIN 0,-35.56; VIN1 -2.54,-35.56
IND_ELL8TP = smd 2.054 x 3.2 rotated 45: 1 -2.442,-2.696; 2 2.442,2.442
SO28W = smd 0.762 x 1.27: 1 -7.62,-4.78; 2 -6.35,-4.78; 3 -5.08,-4.78; 4 -3.81,-4.78; 5 -2.54,-4.78; 6 -1.27,-4.78; 7 0,-4.78; 8 1.27,-4.78; 9 2.54,-4.78; 10 3.81,-4.78; 11 5.08,-4.78; 12 6.35,-4.78; 13 7.62,-4.78; 14 8.89,-4.78; 15 8.89,4.78; 16 7.62,4.78; 17 6.35,4.78; 18 5.08,4.78; 19 3.81,4.78; 20 2.54,4.78; 21 1.27,4.78; 22 0,4.78; 23 -1.27,4.78; 24 -2.54,4.78; 25 -3.81,4.78; 26 -5.08,4.78; 27 -6.35,4.78; 28 -7.62,4.78
SO18L = smd 0.66 x 2.032: 1 -5.08,-4.902; 2 -3.81,-4.902; 3 -2.54,-4.902; 4 -1.27,-4.902; 5 0,-4.902; 6 1.27,-4.902; 7 2.54,-4.902; 8 3.81,-4.902; 9 5.08,-4.902; 10 5.08,4.902; 11 3.81,4.902; 12 2.54,4.902; 13 1.27,4.902; 14 0,4.902; 15 -1.27,4.902; 16 -2.54,4.902; 17 -3.81,4.902; 18 -5.08,4.902
SO-8 = smd 0.6 x 1.55: 1 -1.905,-2.69; 2 -0.635,-2.69; 3 0.635,-2.69; 4 1.905,-2.69; 5 1.905,2.71; 6 0.635,2.71; 7 -0.635,2.71; 8 -1.905,2.71
JUMPER_3X2 = drill 0.9: A1 0,5.08; A2 0,2.54; A3 0,0; B1 2.54,5.08; B2 2.54,2.54; B3 2.54,0
G2R2 = drill 1.321 pad 3.048: 1 -2.54,-3.683; 2 -2.54,3.81; 3 5.08,-3.683; 4 5.08,3.81; O1 12.471,3.81; O2 12.471,-3.683; P1 17.45,3.81; P2 17.45,-3.683; S1 22.454,3.81; S2 22.454,-3.683
CHIPLED_0603 = smd 0.8 x 0.8: A 0,-0.75; C 0,0.75
RNE = smd 0.5 x 0.9: 1 -1.2,-0.8; 2 -0.4,-0.8; 3 0.4,-0.8; 4 1.2,-0.8; 5 1.2,0.8; 6 0.4,0.8; 7 -0.4,0.8; 8 -1.2,0.8
RND = smd 0.5 x 0.9: 1 -1.2,-0.8; 2 -0.4,-0.8; 3 0.4,-0.8; 4 1.2,-0.8; 5 1.2,0.8; 6 0.4,0.8; 7 -0.4,0.8; 8 -1.2,0.8
RNB = smd 0.5 x 0.9: 1 -1.2,-0.8; 2 -0.4,-0.8; 3 0.4,-0.8; 4 1.2,-0.8; 5 1.2,0.8; 6 0.4,0.8; 7 -0.4,0.8; 8 -1.2,0.8
PCB_MOUNTING_HOLE = hole 3.962: 4.445,4.445
PJ-102A = drill 3 pad 4.8: RING 0.1,-3.39; TIP 0.1,-9.29 | drill 3 pad 3.251: RING_SW -4.6,-6.29
MDSTB3 = drill 1.524 pad 3.81: 1 -3.81,-10.795; 2 1.27,-10.795; 3 6.35,-10.795 | drill 1.524 pad 2.54 long: 4 -6.35,5.08; 5 -1.27,5.08; 6 3.81,5.08
70553-04 = drill 1.1 pad 1.778 octagon: 1 -3.81,-7.62; 2 -1.27,-7.62; 3 1.27,-7.62; 4 3.81,-7.62
MKDSN1,5/2-5,08 = drill 1.3 pad 3.048: 1 -2.561,0.025; 2 2.519,0.025

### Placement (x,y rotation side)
BRA2  145.41,58.43 180 top
C1  105.73,72.72 0 top
C4  105.73,77.48 0 top
C6  100.33,77.48 0 top
C7  100.33,72.72 0 top
C9  117.6,74.05 270 top
C10  117.6,65.27 90 top
C17  85.09,62.24 0 top
C20  93.34,62.24 0 top
C22  8.89,91.45 0 top
C23  4.44,50.18 0 top
C24  8.25,104.15 0 top
CD1  112.14,65.67 270 top
D1  125.35,58.94 0 top
FOR_NANO  161.29,91.45 270 top
H1  134.49,61.61 0 top
IC1  88.9,76.21 180 top
IC3  67.94,68.91 180 top
IC4  67.94,83.2 0 top
IC6  124.97,64.27 270 top
JP1  104.78,85.74 0 top
K1  140.97,50.18 270 top
K2  125.73,50.18 270 top
K3  110.49,50.18 270 top
K4  95.25,50.18 270 top
K5  62.86,50.18 270 top
K6  47.62,50.18 270 top
K7  32.38,50.18 270 top
K8  17.14,50.18 270 top
K9  148.59,102.25 90 top
K10  133.35,102.25 90 top
K11  118.11,102.25 90 top
K12  102.87,102.25 90 top
K13  70.48,102.25 90 top
K14  55.25,102.25 90 top
K15  40,102.25 90 top
K16  24.76,102.25 90 top
POWER1  162.88,29.86 180 top
R1  38.1,73.67 180 top
R2  34.29,73.67 180 top
R3  30.48,73.67 180 top
R4  26.67,73.67 180 top
R5  22.86,73.67 180 top
R6  19.05,73.67 180 top
R7  15.24,73.67 180 top
R8  11.43,73.67 180 top
R9  38.1,78.75 0 top
R10  34.29,78.75 0 top
R11  30.48,78.75 0 top
R12  26.67,78.75 0 top
R13  22.86,78.75 0 top
R14  19.05,78.75 0 top
R15  15.24,78.75 0 top
R16  11.43,78.75 0 top
RN1  99.69,88.28 90 top
RN3  134.24,83.83 0 top
RN5  45.72,82.56 270 top
RN6  49.53,82.56 270 top
RN7  49.53,78.75 270 top
RN8  45.72,78.75 270 top
RN9  49.53,69.86 270 top
RN10  45.72,69.86 270 top
RN11  49.53,73.67 90 top
RN12  45.72,73.67 90 top
RN18  105.41,64.78 90 top
RN19  105.41,68.59 90 top
RN20  89.53,92.21 180 top
RN21  94.49,92.21 180 top
RNB1  158.37,29.92 90 top
U$1  87,143.52 90 top
U$5  PCB_MOUNTING_HOLE  [PCB_MOUNTING_HOLE]  165.1,143.52 90 top
U$6  160.66,60.72 270 top
U$7  [ICON_MINUS]  154.94,47.64 90 top
U$8  [ICON_PLUS]  154.94,53.04 0 top
U$9  PCB_MOUNTING_HOLE  [PCB_MOUNTING_HOLE]  8.89,143.52 90 top
U$10  PCB_MOUNTING_HOLE  [PCB_MOUNTING_HOLE]  78.1,8.9 270 top
U$11  PCB_MOUNTING_HOLE  [PCB_MOUNTING_HOLE]  156.21,8.9 270 top
U$12  PCB_MOUNTING_HOLE  [PCB_MOUNTING_HOLE]  0,8.9 270 top
U$15  [VISION_REF15]  162.56,11.44 90 top
U$17  [ICON_MINUS]  154.94,47.64 90 top
U$18  [VISION_REF10]  162.56,140.98 90 top
U$19  [ICON_PLUS]  154.94,53.04 0 top
U$21  [ICON_USA]  163.83,126.38 90 top
U$22  [ICON_MINUS]  154.94,47.64 90 top
U$23  [VISION_REF15]  1.91,141.62 90 top
U$24  [ICON_PLUS]  154.94,53.04 0 top
U$28  [VISION_REF10]  1.91,10.81 90 top
X1  146.05,136.54 180 top
X2  130.81,136.54 180 top
X3  115.57,136.54 180 top
X4  100.33,136.54 180 top
X5  67.94,136.54 180 top
X6  52.7,136.54 180 top
X7  37.47,136.54 180 top
X8  22.22,136.54 180 top
X10  159.13,81.29 270 top
X17  160.66,50.5 90 top
X28  143.51,15.89 0 top
X29  128.27,15.89 0 top
X30  113.03,15.89 0 top
X31  97.79,15.89 0 top
X32  65.41,15.89 0 top
X33  50.16,15.89 0 top
X34  34.92,15.89 0 top
X35  19.69,15.89 0 top

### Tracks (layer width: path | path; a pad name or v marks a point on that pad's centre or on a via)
GND  (via drill 0.5, 0.6, 0.9)
  Top 0.254: 133.35,74.82 133.35,76.85 132.72,77.48 | FOR_NANO.GND@1 133.35,69.86 | 128.27,93.99 128.27,87.01
  Top 0.406: C1.2 C4.2
  Top 1.016: 133.35,67.45 133.35,73.67 133.35,74.82
  Bottom 0.254: 128.27,88.91 FOR_NANO.GND
  other vias: 103.25,87.39 85.72,82.56 118.74,83.2 155.58,83.83 128.91,84.09 159.39,83.83 142.87,80.02 144.27,76.47 125.35,62.62
  pour Top (isolate 0.305): 173.29,43.83 153.35,43.83 153.35,57.16 173.29,57.16
  pour Top (isolate 0.305): -1.91,95.26 165.1,95.26 165.1,57.16 -1.91,57.16
  pour Bottom (isolate 0.305): -3.18,57.16 -3.18,94.63 165.1,95.26 165.1,57.16
  pour Top (isolate 0.305): -2.54,57.16 -2.54,44.46 9.53,44.46 9.53,57.16
  pour Bottom (isolate 0.305): -5.08,44.46 -5.08,57.16 9.53,57.16 9.53,44.46
  pour Bottom (isolate 0.305): -1.91,93.99 -1.91,109.23 17.14,109.23 17.14,93.99
  pour Top (isolate 0.305): -4.45,94.63 -4.45,109.23 17.14,109.23 17.14,94.63
  pour Top (isolate 0.305): 169.23,22.87 153.35,22.87 153.35,55.89 169.23,55.89
  pour Top: 164.78,22.87 153.99,22.87 153.99,55.89 164.78,55.89
I2C_SCL  (via drill 0.5, 0.6, 0.9)
  Top 0.254: v118.74,88.28 111.76,88.28 111.12,87.64 v111.12,78.75 | X10.4 138.05,77.48 138.05,78.12 137.03,79.13 134.87,79.13 134.64,79.37 RN3.3 134.62,83.01 134.62,81.29 v133.98,81.29
  Top 0.305: v82.55,79.39 IC1.12
  Top 0.406: v118.74,88.28 121.92,88.28 122.55,87.64 122.55,84.47 124.46,82.56 v125.73,82.56
  Bottom 0.305: v111.12,78.75 83.19,78.75 v82.55,79.39 | FOR_NANO.A5 140.97,84.47 147.96,77.48 X10.4
  Bottom 0.406: v125.73,82.56 132.72,82.56 v133.98,81.29
I2C_SDA  (via drill 0.5, 0.6, 0.9)
  Top 0.254: v118.74,90.82 111.12,90.82 109.85,89.55 v109.85,77.48 | RN3.4 135.44,82.63 v136.14,81.93 | v136.77,77.47 v136.78,77.48 | X10.3 147.32,80.02 146.05,78.75 v139.06,78.75
  Top 0.305: v81.28,78.12 IC1.13
  Top 0.406: v118.74,90.82 122.55,90.82 123.83,89.55 123.83,87.01 v125.73,85.1
  Bottom 0.254: v136.14,81.93 136.14,78.12 v136.78,77.48 138.05,78.75 v139.06,78.75
  Bottom 0.305: v81.28,78.12 109.22,78.12 v109.85,77.48 | FOR_NANO.A4 143.51,85.1 148.59,80.02 X10.3
  Bottom 0.406: v125.73,85.1 133.37,85.1 RN3.4 135.44,82.63 v136.14,81.93
N$1
  Bottom 1.27: X1.5 149.86,128.92 149.86,122.11 K9.P2
N$2
  Bottom 1.27: X1.6 147.96,125.74 147.96,119.04 K9.O2
N$3
  Top 2.54: X1.4 152.4,124.83 K9.S2
N$4
  Top 1.27: K9.P1 144.47,119.7 141.6,122.57 141.6,125.74 144.78,128.92 144.78,134.63
  Top 2.54: X1.2 144.78,134.63
N$5
  Top 1.27: K9.O1 144.37,114.72 139.7,119.39 139.7,134.63
  Top 2.54: X1.3 139.7,134.63
N$6
  Top 1.27: K9.S1 145.64,124.7 149.86,128.92 149.86,134.63
  Top 2.54: X1.1 149.86,134.63
N$7
  Bottom 1.27: X2.5 134.62,128.92 134.62,122.11 K10.P2
N$8
  Bottom 1.27: X2.6 132.72,125.74 132.72,119.04 K10.O2
N$9
  Top 2.54: X2.4 137.16,124.83 K10.S2
N$10
  Top 1.27: K10.S1 130.4,124.7 134.62,128.92 134.62,134.63
  Top 2.54: X2.1 134.62,134.63
N$11
  Top 1.27: K10.P1 129.23,119.7 126.36,122.57 126.36,125.74 129.54,128.92 129.54,134.63
  Top 2.54: X2.2 129.54,134.63
N$12
  Top 1.27: K10.O1 129.13,114.72 124.46,119.39 124.46,134.63
  Top 2.54: X2.3 124.46,134.63
N$13
  Bottom 1.27: X3.5 119.38,128.92 119.38,122.11 K11.P2
N$14
  Bottom 1.27: X3.6 117.47,125.74 117.47,119.04 K11.O2
N$15
  Bottom 1.27: X4.5 104.14,128.92 104.14,122.11 K12.P2
N$16
  Bottom 1.27: X4.6 102.23,125.74 102.23,119.04 K12.O2
N$17
  Top 2.54: X3.4 121.92,124.83 K11.S2
N$18
  Top 2.54: X4.4 106.68,124.83 K12.S2
N$19
  Top 1.27: K11.O1 113.89,114.72 109.22,119.39 109.22,134.63
  Top 2.54: X3.3 109.22,134.63
N$20
  Top 1.27: K12.O1 98.65,114.72 93.98,119.39 93.98,134.63
  Top 2.54: X4.3 93.98,134.63
N$21
  Top 1.27: K12.P1 98.75,119.7 95.88,122.57 95.88,125.74 99.06,128.92 99.06,134.63
  Top 2.54: X4.2 99.06,134.63
N$22
  Top 1.27: K11.P1 113.99,119.7 111.12,122.57 111.12,125.74 114.3,128.92 114.3,134.63
  Top 2.54: X3.2 114.3,134.63
N$23
  Top 1.27: K11.S1 115.16,124.7 119.38,128.92 119.38,134.63
  Top 2.54: X3.1 119.38,134.63
N$24
  Top 1.27: K12.S1 99.92,124.7 104.14,128.92 104.14,134.63
  Top 2.54: X4.1 104.14,134.63
N$25
  Bottom 1.27: X5.6 69.85,125.74 69.85,119.04 K13.O2
N$26
  Bottom 1.27: X5.5 71.75,128.92 71.75,122.11 K13.P2
N$27
  Top 2.54: X5.4 74.29,124.83 K13.S2
N$28
  Top 1.27: K13.P1 66.37,119.7 63.5,122.57 63.5,125.74 66.67,128.92 66.67,134.63
  Top 2.54: X5.2 66.67,134.63
N$29
  Top 1.27: K13.S1 67.54,124.7 71.75,128.92 71.75,134.63
  Top 2.54: X5.1 71.75,134.63
N$30
  Top 1.27: K13.O1 66.27,114.72 61.59,119.39 61.59,134.63
  Top 2.54: X5.3 61.59,134.63
N$31
  Bottom 1.27: X6.5 56.51,128.92 56.51,122.11 K14.P2
N$32
  Bottom 1.27: X6.6 54.61,125.74 54.61,119.04 K14.O2
N$33
  Top 1.27: K14.P1 51.13,119.7 48.26,122.57 48.26,125.74 51.44,128.92 51.44,134.63
  Top 2.54: X6.2 51.44,134.63
N$34
  Top 1.27: K14.S1 52.3,124.7 56.51,128.92 56.51,134.63
  Top 2.54: X6.1 56.51,134.63
N$35
  Top 1.27: K15.P1 35.89,119.7 33.02,122.57 33.02,125.74 36.19,128.92 36.19,134.63
  Top 2.54: X7.2 36.19,134.63
N$36
  Top 1.27: K16.P1 20.65,119.7 17.78,122.57 17.78,125.74 20.95,128.92 20.95,134.63
  Top 2.54: X8.2 20.95,134.63
N$37
  Bottom 1.27: X8.5 26.03,128.92 26.03,122.11 K16.P2
N$38
  Bottom 1.27: X8.6 24.13,125.74 24.13,119.04 K16.O2
N$39
  Top 1.27: K14.O1 51.44,114.95 46.35,120.03 46.35,134.63
  Top 2.54: X6.3 46.35,134.63
N$40
  Top 1.27: K16.O1 20.55,114.72 15.88,119.39 15.88,134.63
  Top 2.54: X8.3 15.88,134.63
N$41
  Top 1.27: K15.O1 35.79,114.72 31.11,119.39 31.11,134.63
  Top 2.54: X7.3 31.11,134.63
N$42
  Bottom 1.27: X7.6 39.37,125.74 39.37,119.04 K15.O2
N$43
  Bottom 1.27: X7.5 41.28,128.92 41.28,122.11 K15.P2
N$44
  Top 2.54: X6.4 59.05,124.83 K14.S2
N$45
  Top 2.54: X7.4 43.81,124.83 K15.S2
N$46
  Top 1.27: K15.S1 37.06,124.7 41.28,128.92 41.28,134.63
  Top 2.54: X7.1 41.28,134.63
N$47
  Top 1.27: K16.S1 21.82,124.7 26.03,128.92 26.03,134.63
  Top 2.54: X8.1 26.03,134.63
N$48
  Top 2.54: X8.4 28.57,124.83 K16.S2
N$49  (via drill 0.5)
  Top 0.406: JP1.A1 103.89,90.82 101.73,88.66 100.51,88.66 RN1.3 | IC1.15 80.01,73.04 79.38,73.67 77.47,73.67 76.83,74.31 v76.83,77.48
  Bottom 0.406: v76.83,77.48 76.83,83.83 77.47,84.47 83.19,84.47 83.82,85.1 83.82,92.09 84.45,92.72 101.6,92.72 103.7,90.63 104.59,90.63 JP1.A1
N$68
  Bottom 2.54: 160.66,52.72 154.94,52.72 151.13,56.53
N$99
  Top 0.254: POWER1.A 160.9,30.61 160.53,30.24 159.25,30.24 RNB1.3
  Top 0.406: 159.21,30.37 RNB1.3
N$100
  Top 0.813: 126.36,66.18 IC6.8 134.8,66.18 H1.2 | 126.36,66.18 124.59,66.18 123.83,65.42 123.83,60.87 123.32,60.36 123.32,58.96 D1.C 123.17,58.81 121.16,58.81 119.89,60.08 112.65,60.08 112.14,60.59 CD1.2 | 126.34,66.2 126.36,66.18
N$101
  Top 0.813: CD1.1 114.45,67.17 115.57,66.05 120.4,66.05 120.52,66.18 IC6.1
N$203
  Bottom 1.27: X28.5 139.7,23.51 139.7,30.31 K1.P2
N$204
  Bottom 1.27: X28.6 141.6,26.05 141.6,32.75 K1.O2
N$205
  Top 2.54: X28.4 137.16,27.6 K1.S2
N$206
  Top 1.27: K1.P1 145.09,32.73 147.96,29.86 147.96,26.68 144.78,23.51 144.78,17.79
  Top 2.54: X28.2 144.78,17.79
N$207
  Top 1.27: K1.O1 144.78,37.48 149.86,32.4 149.86,17.79
  Top 2.54: X28.3 149.86,17.79
N$208
  Top 1.27: 139.7,17.79 139.7,24.78 142.65,27.72 K1.S1
  Top 2.54: X28.1 139.7,17.79
N$209
  Bottom 1.27: X29.5 124.46,23.51 124.46,30.31 K2.P2
N$210
  Bottom 1.27: X29.6 126.36,26.68 126.36,33.39 K2.O2
N$211
  Top 2.54: X29.4 121.92,27.6 K2.S2
N$212
  Top 1.27: K2.S1 129.54,27.32 127.64,27.32 124.46,24.14 124.46,17.79
  Top 2.54: X29.1 124.46,17.79
N$213
  Top 1.27: K2.P1 129.84,32.73 132.72,29.86 132.72,26.68 129.54,23.51 129.54,17.79
  Top 2.54: X29.2 129.54,17.79
N$214
  Top 1.27: K2.O1 129.54,37.48 134.62,32.4 134.62,17.79
  Top 2.54: X29.3 134.62,17.79
N$215
  Bottom 1.27: X30.5 109.22,23.51 109.22,30.31 K3.P2
N$216
  Bottom 1.27: X30.6 111.12,26.68 111.12,33.39 K3.O2
N$217
  Bottom 1.27: X31.5 95.88,20.97 93.98,22.87 93.98,30.31 K4.P2
N$218
  Bottom 1.27: X31.6 95.88,26.68 95.88,33.39 K4.O2
N$219
  Top 2.54: X30.4 106.68,27.6 K3.S2
N$220
  Top 2.54: X31.4 91.57,20.97 K4.S2
N$221
  Top 1.27: K3.O1 114.71,37.71 119.38,33.03 119.38,17.79
  Top 2.54: X30.3 119.38,17.79
N$222
  Top 1.27: 104.14,17.79 104.14,32.63 K4.O1
  Top 2.54: X31.3 104.14,17.79
N$223
  Top 1.27: K4.P1 99.06,32.4 102.23,29.22 102.23,26.68 99.06,23.51 99.06,17.79
  Top 2.54: 99.06,17.79 X31.2
N$224
  Top 1.27: 114.3,17.79 114.3,23.51 117.47,26.68 117.53,29.48 117.17,29.86 K3.P1
  Top 2.54: X30.2 114.3,17.79
N$225
  Top 1.27: 109.22,17.79 109.22,24.14 112.8,27.72 K3.S1
  Top 2.54: X30.1 109.22,17.79
N$226
  Top 1.27: 93.98,17.79 93.98,24.14 97.56,27.72 K4.S1
  Top 2.54: X31.1 93.98,17.79
N$304
  Bottom 1.27: X32.6 63.5,26.68 63.5,33.39 K5.O2
N$305
  Bottom 1.27: X32.5 61.59,23.51 61.59,30.31 K5.P2
N$306
  Top 2.54: X32.4 59.05,27.6 K5.S2
N$307
  Top 1.27: 66.67,17.79 66.67,23.51 69.85,26.68 69.85,29.55 K5.P1
  Top 2.54: X32.2 66.67,17.79
N$308
  Top 1.27: 61.59,17.79 61.59,24.14 65.18,27.72 K5.S1
  Top 2.54: X32.1 61.59,17.79
N$309
  Top 1.27: 71.75,17.79 71.75,32.63 K5.O1
  Top 2.54: X32.3 71.75,17.79
N$310
  Bottom 1.27: X33.5 46.35,23.51 46.35,30.31 K6.P2
N$311
  Bottom 1.27: X33.6 48.26,26.68 48.26,33.39 K6.O2
N$312
  Top 1.27: 51.44,17.79 51.44,23.51 54.61,26.68 54.61,29.55 K6.P1
  Top 2.54: X33.2 51.44,17.79
N$313
  Top 1.27: 46.35,17.79 46.35,24.14 49.94,27.72 K6.S1
  Top 2.54: X33.1 46.35,17.79
N$314
  Top 1.27: 36.19,17.79 36.19,23.51 39.37,26.68 39.37,29.55 K7.P1
  Top 2.54: X34.2 36.19,17.79
N$315
  Top 1.27: 20.95,17.79 20.95,23.51 24.13,26.68 24.13,29.55 K8.P1
  Top 2.54: X35.2 20.95,17.79
N$316
  Bottom 1.27: X35.5 15.88,23.51 15.88,30.31 K8.P2
N$317
  Bottom 1.27: X35.6 17.78,26.68 17.78,33.39 K8.O2
N$318
  Top 1.27: 56.51,17.79 56.51,32.63 K6.O1
  Top 2.54: X33.3 56.51,17.79
N$319
  Top 1.27: 26.03,17.79 26.03,32.63 K8.O1
  Top 2.54: X35.3 26.03,17.79
N$320
  Top 1.27: 41.28,17.79 41.28,32.63 K7.O1
  Top 2.54: X34.3 41.28,17.79
N$321
  Bottom 1.27: X34.6 33.02,26.68 33.02,33.39 K7.O2
N$322
  Bottom 1.27: X34.5 31.11,23.51 31.11,30.31 K7.P2
N$323
  Top 2.54: X33.4 43.81,27.6 K6.S2
N$324
  Top 2.54: X34.4 28.57,27.6 K7.S2
N$325
  Top 1.27: 31.11,17.79 31.11,24.78 34.06,27.72 K7.S1
  Top 2.54: X34.1 31.11,17.79
N$326
  Top 1.27: 15.88,17.79 15.88,24.14 19.46,27.72 K8.S1
  Top 2.54: X35.1 15.88,17.79
N$327
  Top 2.54: X35.4 13.33,27.6 K8.S2
N$405  (via drill 0.5)
  Top 0.229: IC1.21 87.63,70.81 87,70.18 73.66,70.18 73.03,70.81 IC3.1
  Top 0.254: 87.63,70.81 v87.63,73.29 | v101.85,70.37 102.49,69.74 104.55,69.74
  Top 0.305: 104.55,69.74 104.61,69.74 RN19.5
  Bottom 0.229: v87.63,73.29 87.63,73.04 88.26,73.67 101.22,73.67 101.85,73.04 v101.85,70.37
N$406  (via drill 0.5)
  Top 0.229: IC1.25 v92.71,69.99 92.71,68.28 92.07,67.64 68.58,67.64 67.94,68.28 IC3.5 | v98.42,66.37 101.92,66.37 102.23,66.05 104.54,66.05 RN18.5
  Bottom 0.229: v92.71,69.99 92.71,71.28 93.07,71.64 98.02,71.64 98.43,71.24 v98.42,66.37
N$407  (via drill 0.5)
  Top 0.229: IC1.26 v93.98,69.99 93.98,67.96 93.03,67.01 67.31,67.01 66.67,67.64 IC3.6 | v99.38,65.42 101.92,65.42 102.23,65.1 104.53,65.1 RN18.6
  Bottom 0.229: v93.98,69.99 93.98,71.01 94.11,71.13 97.28,71.13 97.41,71.01 97.41,65.67 97.66,65.42 v99.38,65.42
N$408  (via drill 0.5)
  Top 0.406: JP1.A2 102.36,88.28 101.98,87.9 100.51,87.9 RN1.2 | IC1.16 81.28,73.67 80.01,74.94 78.74,74.94 78.1,75.58 v78.1,76.21
  Bottom 0.406: v78.1,76.21 78.1,83.2 78.74,83.83 83.82,83.83 84.45,84.47 84.45,91.45 85.09,92.09 100.97,92.09 102.23,90.82 102.23,88.91 102.87,88.28 JP1.A2
N$409  (via drill 0.5)
  Top 0.229: IC1.22 88.9,70.18 88.26,69.54 72.39,69.54 71.75,70.18 IC3.2
  Top 0.254: 88.9,70.18 v88.9,69.99 | v100.84,69.61 101.35,69.61 101.98,68.97 104.59,68.97 RN19.6
  Bottom 0.229: v88.9,69.99 88.9,72.78 89.28,73.16 100.33,73.16 100.84,72.66 v100.84,69.61
N$410  (via drill 0.5)
  Top 0.229: IC1.23 90.17,69.54 89.53,68.91 71.12,68.91 70.48,69.54 IC3.3
  Top 0.254: 90.17,69.54 v90.17,69.99 | v99.95,68.59 100.58,68.59 100.97,68.21 104.59,68.21 RN19.7
  Bottom 0.229: v90.17,69.99 90.17,72.4 90.42,72.66 99.57,72.66 99.95,72.28 v99.95,68.59
  Bottom 0.254: 100.2,68.47 v99.95,68.59
N$411  (via drill 0.5)
  Top 0.229: IC1.24 91.44,68.91 90.8,68.28 69.85,68.28 69.22,68.91 IC3.4
  Top 0.254: 91.44,68.91 v91.44,69.99 | v99.57,67.32 104.54,67.32 RN19.8
  Bottom 0.229: v91.44,69.99 91.44,71.64 91.95,72.15 98.3,72.15 99.06,71.39 99.06,67.83 v99.57,67.32
N$416  (via drill 0.6)
  Top 0.203: 71.75,79.39 72.07,79.7 77.79,79.7 78.74,80.66 78.74,82.88 79.38,83.51 95.88,83.51 96.52,84.15 v96.52,88.91
  Top 0.229: v96.52,88.91 96.52,89.8 95.76,90.56 95.76,91.34 RN21.8
  Top 0.406: v96.52,82.56 IC1.1 | IC4.8 71.75,79.39
  Bottom 0.406: v96.52,88.91 v96.52,82.56
N$417  (via drill 0.6)
  Top 0.203: IC4.7 70.48,79.7 70.99,80.21 77.28,80.21 78.1,81.04 78.1,83.51 78.74,84.15 94.61,84.15 95.25,84.78 v95.25,88.91
  Top 0.229: v95.25,88.91 95.25,89.93 94.87,90.31 94.87,91.4 RN21.7
  Top 0.406: v95.25,82.56 IC1.2
  Bottom 0.406: v95.25,88.91 v95.25,82.56
N$418  (via drill 0.6)
  Top 0.203: IC4.6 69.22,80.02 69.91,80.72 76.52,80.72 77.47,81.67 77.47,84.15 78.1,84.78 93.34,84.78 93.98,85.42 v93.98,88.91
  Top 0.229: v93.98,88.91 93.98,90.44 94.11,90.56 94.11,91.4 RN21.6
  Top 0.406: v93.98,82.56 IC1.3
  Bottom 0.406: v93.98,88.91 v93.98,82.56
N$419  (via drill 0.6)
  Top 0.203: IC4.5 67.94,80.02 69.15,81.23 75.88,81.23 76.83,82.18 76.83,84.78 77.47,85.42 92.07,85.42 92.71,86.06 v92.71,88.91
  Top 0.229: v92.71,88.91 92.71,90.06 93.22,90.56 93.22,91.34 RN21.5
  Top 0.406: v92.71,82.56 IC1.4
  Bottom 0.406: v92.71,82.56 v92.71,88.91
N$420  (via drill 0.6)
  Top 0.203: IC4.4 66.67,80.02 68.39,81.74 75.37,81.74 76.2,82.56 76.2,85.42 76.83,86.06 90.8,86.06 91.44,86.69 v91.44,88.91
  Top 0.229: v91.44,88.91 91.44,89.67 90.8,90.31 90.8,91.34 RN20.8
  Top 0.406: v91.44,82.56 IC1.5
  Bottom 0.406: v91.44,88.91 v91.44,82.56
N$421  (via drill 0.6)
  Top 0.203: IC4.3 65.41,80.02 67.63,82.25 74.87,82.25 75.56,82.94 75.56,86.06 76.2,86.69 89.53,86.69 90.17,87.32 v90.17,88.91
  Top 0.229: v90.17,88.91 90.17,90.06 89.92,90.31 89.92,91.4 RN20.7
  Top 0.406: v90.17,82.56 IC1.6
  Bottom 0.406: v90.17,88.91 v90.17,82.56
N$422  (via drill 0.6)
  Top 0.203: IC4.2 64.13,80.02 66.87,82.75 74.23,82.75 74.93,83.45 74.93,86.69 75.56,87.32 88.45,87.32 88.9,87.77 v88.9,88.91
  Top 0.229: IC1.7 88.9,80.66 | v88.9,88.91 88.9,89.93 89.15,90.18 89.15,91.4 RN20.6
  Top 0.406: 88.9,88.54 v88.9,88.91 | v88.9,82.56 IC1.7
  Bottom 0.406: v88.9,88.91 v88.9,82.56
N$423  (via drill 0.6)
  Top 0.203: IC4.1 62.86,80.02 66.23,83.39 73.72,83.39 74.29,83.96 74.29,87.25 75,87.96 87.18,87.96 87.63,88.41 v87.63,88.91
  Top 0.229: v87.63,88.91 87.63,89.93 88.26,90.56 88.26,91.34 RN20.5
  Top 0.406: v87.63,82.56 IC1.8
  Bottom 0.406: v87.63,82.56 v87.63,88.91
N$441
  Top 0.406: RN5.1 43.25,83.76 42.54,84.47 16.39,84.47 R16.C
N$442
  Top 0.406: RN8.7 RN7.2
N$443
  Top 0.406: RN7.3 RN8.6
N$444
  Top 0.406: RN8.5 RN7.4
N$445
  Top 0.406: RN5.2 42.78,82.96 41.91,83.83 19.57,83.83 R15.C
N$447
  Top 0.406: RN5.4 41.84,81.36 40.64,82.56 25.92,82.56 R13.C
N$448
  Top 0.406: RN5.5 RN6.4
N$449
  Top 0.406: RN7.1 RN8.8
N$450
  Top 0.406: RN8.1 41.98,79.95 40,81.93 29.09,81.93 R12.C
N$451
  Top 0.406: RN5.6 RN6.3
N$452
  Top 0.406: RN8.2 41.51,79.15 39.37,81.29 32.27,81.29 R11.C
N$453
  Top 0.406: RN6.2 RN5.7
N$454
  Top 0.406: RN5.8 RN6.1
N$458
  Top 0.406: RN5.3 42.31,82.16 41.28,83.2 22.75,83.2 R14.C
N$459
  Top 0.406: RN8.3 41.04,78.35 38.73,80.66 35.44,80.66 R10.C
N$463
  Top 0.406: RN12.4 RN11.5
N$470
  Top 0.406: RN8.4 40.57,77.55 38.73,79.39 38.22,79.39 R9.C
N$473
  Top 0.406: RN12.5 40.57,74.87 38.73,73.04 38.22,73.04 R1.C
N$474
  Top 0.406: RN11.6 RN12.3
N$475
  Top 0.406: RN12.6 41.04,74.07 38.73,71.77 35.44,71.77 R2.C
N$476
  Top 0.406: RN12.7 41.51,73.27 39.37,71.13 32.27,71.13 R3.C
N$477
  Top 0.406: RN9.4 RN10.5
N$478
  Top 0.406: RN10.6 RN9.3
N$479
  Top 0.406: RN9.2 RN10.7
N$480
  Top 0.406: RN10.8 RN9.1
N$481
  Top 0.406: RN12.2 RN11.7
N$482
  Top 0.406: RN10.1 41.84,71.06 40.64,69.86 25.92,69.86 R5.C
N$483
  Top 0.406: RN12.8 41.98,72.47 40,70.5 29.09,70.5 R4.C
N$484
  Top 0.406: RN10.3 42.78,69.46 41.91,68.59 19.57,68.59 R7.C
N$485
  Top 0.406: RN10.4 43.25,68.66 42.54,67.96 16.39,67.96 R8.C
N$486
  Top 0.406: RN10.2 42.31,70.26 41.28,69.23 22.75,69.23 R6.C
N$498  (via drill 0.5)
  Top 0.406: RN1.1 102.16,87.08 103.5,85.74 JP1.A3 | IC1.17 82.55,74.31 80.64,76.21 v80.01,76.21
  Bottom 0.406: v80.01,76.21 80.01,76.85 79.38,77.48 79.38,81.93 80.01,82.56 83.82,82.56 85.09,83.83 85.09,90.82 85.72,91.45 100.33,91.45 100.97,90.82 100.97,87.01 102.23,85.74 JP1.A3
N$500
  Top 0.406: RN11.8 RN12.1
N$525  (via drill 0.5)
  Top 0.229: IC3.7 65.41,67.01 66.04,66.37 94.3,66.37 95.25,67.32 v95.25,69.99 IC1.27 | v100.33,64.47 104.06,64.47 RN18.7
  Bottom 0.229: v100.33,64.47 95.57,64.47 95.25,64.78 v95.25,69.99
N$526
  Top 0.229: IC1.28 96.52,66.37 | 96.52,66.37 95.88,65.73 64.77,65.73 64.13,66.37 IC3.8 | 96.52,66.37 96.52,64.15 97.16,63.51 104.54,63.51 RN18.8
OC_R1_A  (via drill 0.6)
  Top 0.406: IC3.18 v73.03,62.31 73.03,59.7 73.66,59.07 116.21,59.07 116.84,58.43 116.84,57.16 117.47,56.53 144.15,56.53 144.78,55.89 K1.2 | RN11.4 60.89,74.87 v61.09,74.69
  Bottom 0.406: v61.09,74.69 72.39,74.69 73.03,74.05 v73.03,62.31
OC_R1_B
  Top 0.203: RN7.5 59.76,77.55 66.36,84.15 70.8,84.15 71.75,85.1 IC4.11
  Top 0.406: IC4.11 71.75,92.72 72.39,93.36 83.19,93.36 83.82,93.99 114.93,93.99 117.47,96.53 144.15,96.53 144.78,97.17 K9.2
OC_R2_A  (via drill 0.6)
  Top 0.406: RN11.3 59.29,74.07 v59.69,73.67 | IC3.17 v71.75,62.31 71.8,58.46 72.48,57.8 114.93,57.8 115.57,57.16 115.57,55.89 116.21,55.26 128.91,55.26 129.54,54.62 K2.2
  Bottom 0.406: v59.69,73.67 70.48,73.67 71.75,72.4 v71.75,62.31
OC_R2_B
  Top 0.203: IC4.12 70.48,85.74 69.53,84.78 66.36,84.78 59.92,78.35 RN7.6
  Top 0.406: IC4.12 70.48,93.36 71.12,93.99 82.55,93.99 83.19,94.63 114.3,94.63 117.09,97.42 128.91,97.42 129.54,98.06 K10.2
OC_R3_A  (via drill 0.6)
  Top 0.406: RN11.2 57.55,73.27 v58.42,72.4 | IC3.16 v70.48,62.31 70.48,57.16 71.12,56.53 113.66,56.53 114.3,55.89 K3.2
  Bottom 0.406: v58.42,72.4 69.22,72.4 70.48,71.13 v70.48,62.31
OC_R3_B
  Top 0.203: RN7.7 60.09,79.15 66.36,85.42 68.9,85.42 69.22,85.74 IC4.13
  Top 0.406: IC4.13 69.22,93.99 69.85,94.63 81.91,94.63 82.55,95.26 113.66,95.26 114.3,95.9 K11.2
OC_R4_A  (via drill 0.6)
  Top 0.406: RN11.1 55.81,72.47 v57.15,71.13 | IC3.15 v69.22,62.31 69.22,55.89 69.85,55.26 98.42,55.26 99.06,54.62 K4.2
  Bottom 0.406: v57.15,71.13 67.94,71.13 69.22,69.86 v69.22,62.31
OC_R4_B
  Top 0.203: RN7.8 60.25,79.95 66.36,86.06 67.63,86.06 67.94,86.37 IC4.14
  Top 0.406: IC4.14 67.94,94.63 68.58,95.26 81.28,95.26 81.98,95.96 98.11,95.96 99.06,96.91 K12.2
OC_R5_A  (via drill 0.6)
  Top 0.406: RN9.8 54.68,71.06 55.88,69.86 v60.96,69.86 | IC3.14 v67.94,62.31 67.94,56.53 66.67,55.26 K5.2
  Bottom 0.406: v60.96,69.86 66.67,69.86 67.94,68.59 v67.94,62.31
OC_R5_B
  Top 0.203: IC4.15 66.67,87.01 66.36,86.69 66.04,86.69 60.71,81.36 RN6.5
  Top 0.406: K13.2 IC4.15
OC_R6_A  (via drill 0.6)
  Top 0.406: RN9.7 54.21,70.26 55.88,68.59 v59.69,68.59 | IC3.13 v66.67,62.31 66.67,58.43 65.41,57.16 52.07,57.16 51.44,56.53 K6.2
  Bottom 0.406: v59.69,68.59 65.41,68.59 66.67,67.32 v66.67,62.31
OC_R6_B
  Top 0.203: RN6.6 60.56,82.16 65.41,87.01 IC4.16
  Top 0.406: IC4.16 65.41,95 64.51,95.9 52.33,95.9 51.44,96.8 K14.2
OC_R7_A  (via drill 0.6)
  Top 0.406: RN9.6 53.74,69.46 55.88,67.32 v58.42,67.32 | IC3.12 v65.41,62.31 65.41,59.7 64.13,58.43 36.83,58.43 36.19,57.8 K7.2
  Bottom 0.406: v58.42,67.32 64.13,67.32 65.41,66.05 v65.41,62.31
OC_R7_B
  Top 0.203: 60.41,82.96 64.13,86.69 IC4.17
  Top 0.229: 60.41,82.96 RN6.7
  Top 0.406: IC4.17 64.13,93.36 63.5,93.99 36.83,93.99 36.19,94.63 K15.2
OC_R8_A  (via drill 0.6)
  Top 0.406: RN9.5 53.27,68.66 55.88,66.05 v57.15,66.05 | IC3.11 v64.13,62.31 64.13,60.97 62.86,59.7 22.22,59.7 20.95,58.43 K8.2
  Bottom 0.406: v57.15,66.05 62.86,66.05 64.13,64.78 v64.13,62.31
OC_R8_B
  Top 0.203: 60.25,83.76 62.86,86.37 IC4.18
  Top 0.229: 60.25,83.76 RN6.8
  Top 0.406: IC4.18 62.86,92.09 62.23,92.72 21.59,92.72 20.95,93.36 K16.2
REG_5V  (via drill 0.5, 0.6, 0.9)
  Top 0.254: 157.53,30.37 156.34,30.37 v155.58,31.13 | RN3.6 RN3.5 135.51,84.7 135.51,85.23 135.13,85.61 v135.13,85.99
  Top 0.305: 83.82,77.48 85.09,78.75 85.72,78.75 86.36,79.39 | IC1.18 v83.82,76.85 | IC1.9 86.36,79.39 | 86.36,79.39 87,78.75 97.47,78.75 97.79,78.75 | 157.53,30.37 RNB1.6
  Top 0.406: C4.1 C1.1 | C6.1 C7.1 98.83,77.71
  Top 0.61: v135.13,85.99 136.91,85.99 140.34,82.56 X10.2
  Top 0.813: H1.1 130.02,60.18 v129.54,59.7 | IC6.4 120.78,62.37 | 120.78,62.37 v120.65,62.24 | 120.78,62.37 117.71,62.37 C10.1
  Top 1.016: 98.83,77.71 97.79,78.75 | JP1.B3 107.31,83.2 103.82,79.7
  Top 1.27: 97.47,78.75 86.68,78.75 86.36,79.07 85.41,79.07 83.82,77.48 v83.82,76.85 | 98.83,77.71 98.83,79.16 99.69,80.02 103.5,80.02 103.82,79.7 104.14,79.39 104.14,77.57 C4.1 | H1.1 138.53,58.91 v139.06,59.32
  Bottom 0.254: v155.58,31.13 155.58,42.56 156.84,43.83 161.29,43.83 162.56,45.1 162.56,66.69 163.19,67.32 163.19,81.93 162.56,82.56 v157.86,82.56
  Bottom 0.406: JP1.B1 JP1.B2 JP1.B3
  Bottom 0.61: FOR_NANO.5V 133.35,87.77 | 133.35,87.77 v135.13,85.99 | 133.35,87.77 133.35,87.64 132.72,87.01 121.28,87.01 120.02,85.74
  Bottom 0.813: v129.54,59.7 120.65,59.7 v120.65,62.24 119.38,63.51 119.38,74.31 120.65,75.58 120.65,85.1 120.02,85.74 v118.74,85.74
  Bottom 1.016: v157.86,82.56 X10.2 | v118.74,85.74 JP1.B3 | C17.+ v83.82,76.85
REG_12V  (via drill 0.5)
  Top 0.813: BRA2.+ 145.41,63.51 143.51,60.97 135.89,60.97 132.08,64.78 129.79,64.78 v125.6,64.91 IC6.7 | C9.1 117.6,74.82 118.74,73.67 120.02,73.67 120.65,73.04 v120.65,67.96
  Top 1.016: v114.43,77.1 117.55,77.1 C9.1
  Bottom 0.813: v120.65,67.96 120.65,66.05 121.79,64.91 v125.6,64.91
  Bottom 1.016: C20.+ 92.07,60.21 92.96,59.32 105.66,59.32 109.22,62.88 109.22,68.59 113.03,72.4 113.03,75.7 v114.43,77.1
UNREG_12V  (via drill 0.6)
  Top 0.305: 38.1,76.21 R1.A
  Top 0.406: IC4.10 v73.03,86.06 | R8.A 11.43,76.21 | R15.A 15.24,76.21 | R6.A 19.05,76.21 | 22.86,76.21 R13.A | R4.A 26.67,76.21 | R3.A 30.48,76.21 | R2.A 34.29,76.21 | R16.A 11.43,76.21 | 11.43,76.21 15.24,76.21 | R7.A 15.24,76.21 | 15.24,76.21 19.05,76.21 | R14.A 19.05,76.21 | 19.05,76.21 22.86,76.21 | R5.A 22.86,76.21 | 22.86,76.21 26.67,76.21 | R12.A 26.67,76.21 | 26.67,76.21 30.48,76.21 | R11.A 30.48,76.21 | 30.48,76.21 34.29,76.21 | R10.A 34.29,76.21 | R9.A 38.1,76.21 | 38.1,74.31 38.1,76.21 | 38.1,76.21 35.88,76.21 | 34.29,76.21 35.88,76.21 | 35.88,76.21 v35.88,73.04 | IC3.10 62.86,62.88 v62.83,62.31
  Top 2.54: BRA2.~@2 BRA2.~@1 149.18,58.43 U$6.TIP 151.77,60.22 151.77,55.89 154.94,52.72 160.33,52.72 X17.2
  Bottom 0.406: v73.03,86.06 73.03,94.63 72.39,95.26 | v35.88,73.04 35.88,57.16 29.34,57.16 28.7,56.53 | 47.69,57.48 48.01,57.16
  Bottom 1.016: 47.69,57.48 62.83,57.48 v62.83,62.31 | C23.+ 3.17,57.16 | C24.+ 6.98,95.26 | 150.52,56.82 150.52,57.14 150.49,57.16
  Bottom 1.422: C22.+ 7.62,95.26
  Bottom 2.54: 137.16,57.16 150.49,57.16 151.13,57.16 151.13,60.38 U$6.TIP | 137.16,57.16 121.92,57.16 | 121.92,57.16 106.68,57.16 | 106.68,57.16 91.44,57.16 | 91.44,57.16 58.42,57.16 | 58.42,57.16 48.01,57.16 43.81,57.16 | 43.81,57.16 35.88,57.16 13.33,57.16 | 13.33,57.16 3.17,57.16 2.54,57.16 2.54,95.26 6.98,95.26 7.62,95.26 11.43,95.26 | 11.43,95.26 43.81,95.26 | 43.81,95.26 59.05,95.26 | 59.05,95.26 72.39,95.26 74.29,95.26 | 74.29,95.26 89.53,95.26 | 89.53,95.26 106.68,95.26 | 106.68,95.26 121.92,95.26 | 2.41,95.39 11.43,95.26 | K8.1 13.46,57.04 13.33,57.16 | K7.1 28.7,56.53 28.7,57.04 28.57,57.16 | K6.1 43.94,57.04 43.81,57.16 | K5.1 59.18,56.4 58.42,57.16 | K4.1 91.57,57.04 91.44,57.16 | K3.1 106.81,57.04 106.68,57.16 | K2.1 122.05,57.04 121.92,57.16 | K1.1 137.29,57.04 137.16,57.16 | 152.4,99.58 K9.1 152.27,97.68 151.13,96.53 137.16,96.53 | K16.1 28.45,95.39 43.81,95.26 | K15.1 43.69,95.39 59.05,95.26 | K14.1 58.93,95.39 74.29,95.26 | K13.1 74.17,95.39 89.53,95.26 | K12.1 106.55,95.39 106.68,95.26 | K11.1 121.79,95.39 121.92,95.26 | 137.16,96.53 137.16,99.58 K10.1 137.03,96.66 137.16,96.53 | 137.16,96.53 123.19,96.53 121.92,95.26

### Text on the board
tNames: 8 | 5 | 4 | 1 | Bank 2 | ANSR16xDPDT | MCP23017 | REV.E | Address: | A0 | A1 | GND | A2 | +5V | SC | SDA | SCL | 12V DC / Power / Supply | 12V DC / Power / Supply | 12V DC / Power / Supply | 2016 ControlEverything.com | Bank 1 | 8 | 5 | 4 | 1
